DATA_BLOCK "IMAC_MOTOR3_RECORD"
TITLE =  MOTOR3_RECORD
AUTHOR : HottendU
FAMILY : IMAC
VERSION : 0.2


  STRUCT
   MOTOR3_No001 : STRUCT
    System : WORD ;
    CmdOS : WORD ;
    MirrorCmdOS : WORD ;
    Test : WORD ;
    AlarmOS : WORD ;
    StatusOS : WORD ;
    SysStatusOS : WORD ;
    Status1 : WORD ;
    Status2 : WORD ;
    Status3 : BYTE ;
    InputEdges : BYTE ;
    AutoEdges : WORD ;
    DataTimeExtFault : STRUCT
     StartTime : DINT ;
     StartEdge : BOOL ;
    END_STRUCT ;
    DataTimeFeedback : STRUCT
     StartTime : DINT ;
     StartEdge : BOOL ;
    END_STRUCT ;
    DataTimeActFault : STRUCT
     StartTime : DINT ;
     StartEdge : BOOL ;
    END_STRUCT ;
    DataTimeAutoAl : STRUCT
     StartTime : DINT ;
     StartEdge : BOOL ;
    END_STRUCT ;
    DataTimeRestart : STRUCT
     StartTime : DINT ;
     StartEdge : BOOL ;
    END_STRUCT ;
    DataTimeChgSF : STRUCT
     StartTime : DINT ;
     StartEdge : BOOL ;
    END_STRUCT ;
    DataTimeChgFS : STRUCT
     StartTime : DINT ;
     StartEdge : BOOL ;
    END_STRUCT ;
    DataTimeChgDirec : STRUCT
     StartTime : DINT ;
     StartEdge : BOOL ;
    END_STRUCT ;
    PCONF : STRUCT 	//// PCONF MOTOR3 - Instance 001
     Modeswitches : STRUCT
      M0_ConstantOut : BOOL  := TRUE;	// Constant Output MST1 MST2 MSTO (1); Feedback depended Output Anst. (0)
      M1_AutoManLoc : BOOL  := TRUE;	// AUTO/ MANUAL/ LOCAL (1); MANUAL/ LOCAL (0)
      M2_NoActFeedFault : BOOL ;	// No Action- and Non-Feedback fault(1),
      M3_NoStopIfFault : BOOL  := TRUE;	// No Stop-Signal if Failure occurs (1)
      M4_RestrtAftBlack : BOOL  := TRUE;	// Restart after Blackout (1)
      M5_ResetOSonly : BOOL  := TRUE;	// Reset Alarm only with RESET from OS (1); RESET and START/STOP-Command (0)
      sw06 : BOOL ;
      M7_ChgSFviaStop : BOOL ;	// Change from Slow->Fast via STOP(1)
      M8_ChgFSviaStop : BOOL ;	// Change from Fast->Slow via STOP(1)
      M9_StopIfAutoFail : BOOL ;	// Direct Stop if Auto Failure (1)
      M10_ExtFaultNC : BOOL ;	// External Fault is NC (1)
      sw11 : BOOL ;
      sw12 : BOOL ;
      sw13 : BOOL ;
      sw14 : BOOL ;
      sw15 : BOOL ;	//
     END_STRUCT ;
     DlyTExtFault : TIME  := T#1S;	// Setpoint external fault delay
     DlyTFeedback : TIME  := T#1S;	// Setpoint feedback fault delay
     DlyTActFault : TIME  := T#5S;	// Setpoint Action Fault delay
     DlyTAutoAl : TIME  := T#1S;	// Setpoint auto alarm delay
     DlyTRestart : TIME  := T#40S;	// Setpoint restart after blackout delay
     DlyTChgSF : TIME  := T#1S;	// Setpoint Waiting Delay Slow->Fast
     DlyTChgFS : TIME  := T#2S;	// Setpoint Waiting Delay Fast->Slow
     DlyTChgDirec : TIME  := T#4S;	// Setpoint change direction
    END_STRUCT ;
   END_STRUCT ;
   MOTOR3_No002 : STRUCT
    System : WORD ;
    CmdOS : WORD ;
    MirrorCmdOS : WORD ;
    Test : WORD ;
    AlarmOS : WORD ;
    StatusOS : WORD ;
    SysStatusOS : WORD ;
    Status1 : WORD ;
    Status2 : WORD ;
    Status3 : BYTE ;
    InputEdges : BYTE ;
    AutoEdges : WORD ;
    DataTimeExtFault : STRUCT
     StartTime : DINT ;
     StartEdge : BOOL ;
    END_STRUCT ;
    DataTimeFeedback : STRUCT
     StartTime : DINT ;
     StartEdge : BOOL ;
    END_STRUCT ;
    DataTimeActFault : STRUCT
     StartTime : DINT ;
     StartEdge : BOOL ;
    END_STRUCT ;
    DataTimeAutoAl : STRUCT
     StartTime : DINT ;
     StartEdge : BOOL ;
    END_STRUCT ;
    DataTimeRestart : STRUCT
     StartTime : DINT ;
     StartEdge : BOOL ;
    END_STRUCT ;
    DataTimeChgSF : STRUCT
     StartTime : DINT ;
     StartEdge : BOOL ;
    END_STRUCT ;
    DataTimeChgFS : STRUCT
     StartTime : DINT ;
     StartEdge : BOOL ;
    END_STRUCT ;
    DataTimeChgDirec : STRUCT
     StartTime : DINT ;
     StartEdge : BOOL ;
    END_STRUCT ;
    PCONF : STRUCT 	//// PCONF MOTOR3 - Instance 002
     Modeswitches : STRUCT
      M0_ConstantOut : BOOL ;	// Constant Output MST1 MST2 MSTO (1); Feedback depended Output Anst. (0)
      M1_AutoManLoc : BOOL ;	// AUTO/ MANUAL/ LOCAL (1); MANUAL/ LOCAL (0)
      M2_NoActFeedFault : BOOL ;	// No Action- and Non-Feedback fault(1),
      M3_NoStopIfFault : BOOL ;	// No Stop-Signal if Failure occurs (1)
      M4_RestrtAftBlack : BOOL ;	// Restart after Blackout (1)
      M5_ResetOSonly : BOOL ;	// Reset Alarm only with RESET from OS (1); RESET and START/STOP-Command (0)
      sw06 : BOOL ;
      M7_ChgSFviaStop : BOOL ;	// Change from Slow->Fast via STOP(1)
      M8_ChgFSviaStop : BOOL ;	// Change from Fast->Slow via STOP(1)
      M9_StopIfAutoFail : BOOL ;	// Direct Stop if Auto Failure (1)
      M10_ExtFaultNC : BOOL ;	// External Fault is NC (1)
      sw11 : BOOL ;
      sw12 : BOOL ;
      sw13 : BOOL ;
      sw14 : BOOL ;
      sw15 : BOOL ;	//
     END_STRUCT ;
     DlyTExtFault : TIME ;	// Setpoint external fault delay
     DlyTFeedback : TIME ;	// Setpoint feedback fault delay
     DlyTActFault : TIME ;	// Setpoint Action Fault delay
     DlyTAutoAl : TIME ;	// Setpoint auto alarm delay
     DlyTRestart : TIME ;	// Setpoint restart after blackout delay
     DlyTChgSF : TIME ;	// Setpoint Waiting Delay Slow->Fast
     DlyTChgFS : TIME ;	// Setpoint Waiting Delay Fast->Slow
     DlyTChgDirec : TIME ;	// Setpoint change direction
    END_STRUCT ;
   END_STRUCT ;
   MOTOR3_No003 : STRUCT
    System : WORD ;
    CmdOS : WORD ;
    MirrorCmdOS : WORD ;
    Test : WORD ;
    AlarmOS : WORD ;
    StatusOS : WORD ;
    SysStatusOS : WORD ;
    Status1 : WORD ;
    Status2 : WORD ;
    Status3 : BYTE ;
    InputEdges : BYTE ;
    AutoEdges : WORD ;
    DataTimeExtFault : STRUCT
     StartTime : DINT ;
     StartEdge : BOOL ;
    END_STRUCT ;
    DataTimeFeedback : STRUCT
     StartTime : DINT ;
     StartEdge : BOOL ;
    END_STRUCT ;
    DataTimeActFault : STRUCT
     StartTime : DINT ;
     StartEdge : BOOL ;
    END_STRUCT ;
    DataTimeAutoAl : STRUCT
     StartTime : DINT ;
     StartEdge : BOOL ;
    END_STRUCT ;
    DataTimeRestart : STRUCT
     StartTime : DINT ;
     StartEdge : BOOL ;
    END_STRUCT ;
    DataTimeChgSF : STRUCT
     StartTime : DINT ;
     StartEdge : BOOL ;
    END_STRUCT ;
    DataTimeChgFS : STRUCT
     StartTime : DINT ;
     StartEdge : BOOL ;
    END_STRUCT ;
    DataTimeChgDirec : STRUCT
     StartTime : DINT ;
     StartEdge : BOOL ;
    END_STRUCT ;
    PCONF : STRUCT 	//// PCONF MOTOR3 - Instance 003
     Modeswitches : STRUCT
      M0_ConstantOut : BOOL ;	// Constant Output MST1 MST2 MSTO (1); Feedback depended Output Anst. (0)
      M1_AutoManLoc : BOOL ;	// AUTO/ MANUAL/ LOCAL (1); MANUAL/ LOCAL (0)
      M2_NoActFeedFault : BOOL ;	// No Action- and Non-Feedback fault(1),
      M3_NoStopIfFault : BOOL ;	// No Stop-Signal if Failure occurs (1)
      M4_RestrtAftBlack : BOOL ;	// Restart after Blackout (1)
      M5_ResetOSonly : BOOL ;	// Reset Alarm only with RESET from OS (1); RESET and START/STOP-Command (0)
      sw06 : BOOL ;
      M7_ChgSFviaStop : BOOL ;	// Change from Slow->Fast via STOP(1)
      M8_ChgFSviaStop : BOOL ;	// Change from Fast->Slow via STOP(1)
      M9_StopIfAutoFail : BOOL ;	// Direct Stop if Auto Failure (1)
      M10_ExtFaultNC : BOOL ;	// External Fault is NC (1)
      sw11 : BOOL ;
      sw12 : BOOL ;
      sw13 : BOOL ;
      sw14 : BOOL ;
      sw15 : BOOL ;	//
     END_STRUCT ;
     DlyTExtFault : TIME ;	// Setpoint external fault delay
     DlyTFeedback : TIME ;	// Setpoint feedback fault delay
     DlyTActFault : TIME ;	// Setpoint Action Fault delay
     DlyTAutoAl : TIME ;	// Setpoint auto alarm delay
     DlyTRestart : TIME ;	// Setpoint restart after blackout delay
     DlyTChgSF : TIME ;	// Setpoint Waiting Delay Slow->Fast
     DlyTChgFS : TIME ;	// Setpoint Waiting Delay Fast->Slow
     DlyTChgDirec : TIME ;	// Setpoint change direction
    END_STRUCT ;
   END_STRUCT ;
   MOTOR3_No004 : STRUCT
    System : WORD ;
    CmdOS : WORD ;
    MirrorCmdOS : WORD ;
    Test : WORD ;
    AlarmOS : WORD ;
    StatusOS : WORD ;
    SysStatusOS : WORD ;
    Status1 : WORD ;
    Status2 : WORD ;
    Status3 : BYTE ;
    InputEdges : BYTE ;
    AutoEdges : WORD ;
    DataTimeExtFault : STRUCT
     StartTime : DINT ;
     StartEdge : BOOL ;
    END_STRUCT ;
    DataTimeFeedback : STRUCT
     StartTime : DINT ;
     StartEdge : BOOL ;
    END_STRUCT ;
    DataTimeActFault : STRUCT
     StartTime : DINT ;
     StartEdge : BOOL ;
    END_STRUCT ;
    DataTimeAutoAl : STRUCT
     StartTime : DINT ;
     StartEdge : BOOL ;
    END_STRUCT ;
    DataTimeRestart : STRUCT
     StartTime : DINT ;
     StartEdge : BOOL ;
    END_STRUCT ;
    DataTimeChgSF : STRUCT
     StartTime : DINT ;
     StartEdge : BOOL ;
    END_STRUCT ;
    DataTimeChgFS : STRUCT
     StartTime : DINT ;
     StartEdge : BOOL ;
    END_STRUCT ;
    DataTimeChgDirec : STRUCT
     StartTime : DINT ;
     StartEdge : BOOL ;
    END_STRUCT ;
    PCONF : STRUCT 	//// PCONF MOTOR3 - Instance 004
     Modeswitches : STRUCT
      M0_ConstantOut : BOOL ;	// Constant Output MST1 MST2 MSTO (1); Feedback depended Output Anst. (0)
      M1_AutoManLoc : BOOL ;	// AUTO/ MANUAL/ LOCAL (1); MANUAL/ LOCAL (0)
      M2_NoActFeedFault : BOOL ;	// No Action- and Non-Feedback fault(1),
      M3_NoStopIfFault : BOOL ;	// No Stop-Signal if Failure occurs (1)
      M4_RestrtAftBlack : BOOL ;	// Restart after Blackout (1)
      M5_ResetOSonly : BOOL ;	// Reset Alarm only with RESET from OS (1); RESET and START/STOP-Command (0)
      sw06 : BOOL ;
      M7_ChgSFviaStop : BOOL ;	// Change from Slow->Fast via STOP(1)
      M8_ChgFSviaStop : BOOL ;	// Change from Fast->Slow via STOP(1)
      M9_StopIfAutoFail : BOOL ;	// Direct Stop if Auto Failure (1)
      M10_ExtFaultNC : BOOL ;	// External Fault is NC (1)
      sw11 : BOOL ;
      sw12 : BOOL ;
      sw13 : BOOL ;
      sw14 : BOOL ;
      sw15 : BOOL ;	//
     END_STRUCT ;
     DlyTExtFault : TIME ;	// Setpoint external fault delay
     DlyTFeedback : TIME ;	// Setpoint feedback fault delay
     DlyTActFault : TIME ;	// Setpoint Action Fault delay
     DlyTAutoAl : TIME ;	// Setpoint auto alarm delay
     DlyTRestart : TIME ;	// Setpoint restart after blackout delay
     DlyTChgSF : TIME ;	// Setpoint Waiting Delay Slow->Fast
     DlyTChgFS : TIME ;	// Setpoint Waiting Delay Fast->Slow
     DlyTChgDirec : TIME ;	// Setpoint change direction
    END_STRUCT ;
   END_STRUCT ;
   MOTOR3_No005 : STRUCT
    System : WORD ;
    CmdOS : WORD ;
    MirrorCmdOS : WORD ;
    Test : WORD ;
    AlarmOS : WORD ;
    StatusOS : WORD ;
    SysStatusOS : WORD ;
    Status1 : WORD ;
    Status2 : WORD ;
    Status3 : BYTE ;
    InputEdges : BYTE ;
    AutoEdges : WORD ;
    DataTimeExtFault : STRUCT
     StartTime : DINT ;
     StartEdge : BOOL ;
    END_STRUCT ;
    DataTimeFeedback : STRUCT
     StartTime : DINT ;
     StartEdge : BOOL ;
    END_STRUCT ;
    DataTimeActFault : STRUCT
     StartTime : DINT ;
     StartEdge : BOOL ;
    END_STRUCT ;
    DataTimeAutoAl : STRUCT
     StartTime : DINT ;
     StartEdge : BOOL ;
    END_STRUCT ;
    DataTimeRestart : STRUCT
     StartTime : DINT ;
     StartEdge : BOOL ;
    END_STRUCT ;
    DataTimeChgSF : STRUCT
     StartTime : DINT ;
     StartEdge : BOOL ;
    END_STRUCT ;
    DataTimeChgFS : STRUCT
     StartTime : DINT ;
     StartEdge : BOOL ;
    END_STRUCT ;
    DataTimeChgDirec : STRUCT
     StartTime : DINT ;
     StartEdge : BOOL ;
    END_STRUCT ;
    PCONF : STRUCT 	//// PCONF MOTOR3 - Instance 005
     Modeswitches : STRUCT
      M0_ConstantOut : BOOL ;	// Constant Output MST1 MST2 MSTO (1); Feedback depended Output Anst. (0)
      M1_AutoManLoc : BOOL ;	// AUTO/ MANUAL/ LOCAL (1); MANUAL/ LOCAL (0)
      M2_NoActFeedFault : BOOL ;	// No Action- and Non-Feedback fault(1),
      M3_NoStopIfFault : BOOL ;	// No Stop-Signal if Failure occurs (1)
      M4_RestrtAftBlack : BOOL ;	// Restart after Blackout (1)
      M5_ResetOSonly : BOOL ;	// Reset Alarm only with RESET from OS (1); RESET and START/STOP-Command (0)
      sw06 : BOOL ;
      M7_ChgSFviaStop : BOOL ;	// Change from Slow->Fast via STOP(1)
      M8_ChgFSviaStop : BOOL ;	// Change from Fast->Slow via STOP(1)
      M9_StopIfAutoFail : BOOL ;	// Direct Stop if Auto Failure (1)
      M10_ExtFaultNC : BOOL ;	// External Fault is NC (1)
      sw11 : BOOL ;
      sw12 : BOOL ;
      sw13 : BOOL ;
      sw14 : BOOL ;
      sw15 : BOOL ;	//
     END_STRUCT ;
     DlyTExtFault : TIME ;	// Setpoint external fault delay
     DlyTFeedback : TIME ;	// Setpoint feedback fault delay
     DlyTActFault : TIME ;	// Setpoint Action Fault delay
     DlyTAutoAl : TIME ;	// Setpoint auto alarm delay
     DlyTRestart : TIME ;	// Setpoint restart after blackout delay
     DlyTChgSF : TIME ;	// Setpoint Waiting Delay Slow->Fast
     DlyTChgFS : TIME ;	// Setpoint Waiting Delay Fast->Slow
     DlyTChgDirec : TIME ;	// Setpoint change direction
    END_STRUCT ;
   END_STRUCT ;
   MOTOR3_No006 : STRUCT
    System : WORD ;
    CmdOS : WORD ;
    MirrorCmdOS : WORD ;
    Test : WORD ;
    AlarmOS : WORD ;
    StatusOS : WORD ;
    SysStatusOS : WORD ;
    Status1 : WORD ;
    Status2 : WORD ;
    Status3 : BYTE ;
    InputEdges : BYTE ;
    AutoEdges : WORD ;
    DataTimeExtFault : STRUCT
     StartTime : DINT ;
     StartEdge : BOOL ;
    END_STRUCT ;
    DataTimeFeedback : STRUCT
     StartTime : DINT ;
     StartEdge : BOOL ;
    END_STRUCT ;
    DataTimeActFault : STRUCT
     StartTime : DINT ;
     StartEdge : BOOL ;
    END_STRUCT ;
    DataTimeAutoAl : STRUCT
     StartTime : DINT ;
     StartEdge : BOOL ;
    END_STRUCT ;
    DataTimeRestart : STRUCT
     StartTime : DINT ;
     StartEdge : BOOL ;
    END_STRUCT ;
    DataTimeChgSF : STRUCT
     StartTime : DINT ;
     StartEdge : BOOL ;
    END_STRUCT ;
    DataTimeChgFS : STRUCT
     StartTime : DINT ;
     StartEdge : BOOL ;
    END_STRUCT ;
    DataTimeChgDirec : STRUCT
     StartTime : DINT ;
     StartEdge : BOOL ;
    END_STRUCT ;
    PCONF : STRUCT 	//// PCONF MOTOR3 - Instance 006
     Modeswitches : STRUCT
      M0_ConstantOut : BOOL ;	// Constant Output MST1 MST2 MSTO (1); Feedback depended Output Anst. (0)
      M1_AutoManLoc : BOOL ;	// AUTO/ MANUAL/ LOCAL (1); MANUAL/ LOCAL (0)
      M2_NoActFeedFault : BOOL ;	// No Action- and Non-Feedback fault(1),
      M3_NoStopIfFault : BOOL ;	// No Stop-Signal if Failure occurs (1)
      M4_RestrtAftBlack : BOOL ;	// Restart after Blackout (1)
      M5_ResetOSonly : BOOL ;	// Reset Alarm only with RESET from OS (1); RESET and START/STOP-Command (0)
      sw06 : BOOL ;
      M7_ChgSFviaStop : BOOL ;	// Change from Slow->Fast via STOP(1)
      M8_ChgFSviaStop : BOOL ;	// Change from Fast->Slow via STOP(1)
      M9_StopIfAutoFail : BOOL ;	// Direct Stop if Auto Failure (1)
      M10_ExtFaultNC : BOOL ;	// External Fault is NC (1)
      sw11 : BOOL ;
      sw12 : BOOL ;
      sw13 : BOOL ;
      sw14 : BOOL ;
      sw15 : BOOL ;	//
     END_STRUCT ;
     DlyTExtFault : TIME ;	// Setpoint external fault delay
     DlyTFeedback : TIME ;	// Setpoint feedback fault delay
     DlyTActFault : TIME ;	// Setpoint Action Fault delay
     DlyTAutoAl : TIME ;	// Setpoint auto alarm delay
     DlyTRestart : TIME ;	// Setpoint restart after blackout delay
     DlyTChgSF : TIME ;	// Setpoint Waiting Delay Slow->Fast
     DlyTChgFS : TIME ;	// Setpoint Waiting Delay Fast->Slow
     DlyTChgDirec : TIME ;	// Setpoint change direction
    END_STRUCT ;
   END_STRUCT ;
   MOTOR3_No007 : STRUCT
    System : WORD ;
    CmdOS : WORD ;
    MirrorCmdOS : WORD ;
    Test : WORD ;
    AlarmOS : WORD ;
    StatusOS : WORD ;
    SysStatusOS : WORD ;
    Status1 : WORD ;
    Status2 : WORD ;
    Status3 : BYTE ;
    InputEdges : BYTE ;
    AutoEdges : WORD ;
    DataTimeExtFault : STRUCT
     StartTime : DINT ;
     StartEdge : BOOL ;
    END_STRUCT ;
    DataTimeFeedback : STRUCT
     StartTime : DINT ;
     StartEdge : BOOL ;
    END_STRUCT ;
    DataTimeActFault : STRUCT
     StartTime : DINT ;
     StartEdge : BOOL ;
    END_STRUCT ;
    DataTimeAutoAl : STRUCT
     StartTime : DINT ;
     StartEdge : BOOL ;
    END_STRUCT ;
    DataTimeRestart : STRUCT
     StartTime : DINT ;
     StartEdge : BOOL ;
    END_STRUCT ;
    DataTimeChgSF : STRUCT
     StartTime : DINT ;
     StartEdge : BOOL ;
    END_STRUCT ;
    DataTimeChgFS : STRUCT
     StartTime : DINT ;
     StartEdge : BOOL ;
    END_STRUCT ;
    DataTimeChgDirec : STRUCT
     StartTime : DINT ;
     StartEdge : BOOL ;
    END_STRUCT ;
    PCONF : STRUCT 	//// PCONF MOTOR3 - Instance 007
     Modeswitches : STRUCT
      M0_ConstantOut : BOOL ;	// Constant Output MST1 MST2 MSTO (1); Feedback depended Output Anst. (0)
      M1_AutoManLoc : BOOL ;	// AUTO/ MANUAL/ LOCAL (1); MANUAL/ LOCAL (0)
      M2_NoActFeedFault : BOOL ;	// No Action- and Non-Feedback fault(1),
      M3_NoStopIfFault : BOOL ;	// No Stop-Signal if Failure occurs (1)
      M4_RestrtAftBlack : BOOL ;	// Restart after Blackout (1)
      M5_ResetOSonly : BOOL ;	// Reset Alarm only with RESET from OS (1); RESET and START/STOP-Command (0)
      sw06 : BOOL ;
      M7_ChgSFviaStop : BOOL ;	// Change from Slow->Fast via STOP(1)
      M8_ChgFSviaStop : BOOL ;	// Change from Fast->Slow via STOP(1)
      M9_StopIfAutoFail : BOOL ;	// Direct Stop if Auto Failure (1)
      M10_ExtFaultNC : BOOL ;	// External Fault is NC (1)
      sw11 : BOOL ;
      sw12 : BOOL ;
      sw13 : BOOL ;
      sw14 : BOOL ;
      sw15 : BOOL ;	//
     END_STRUCT ;
     DlyTExtFault : TIME ;	// Setpoint external fault delay
     DlyTFeedback : TIME ;	// Setpoint feedback fault delay
     DlyTActFault : TIME ;	// Setpoint Action Fault delay
     DlyTAutoAl : TIME ;	// Setpoint auto alarm delay
     DlyTRestart : TIME ;	// Setpoint restart after blackout delay
     DlyTChgSF : TIME ;	// Setpoint Waiting Delay Slow->Fast
     DlyTChgFS : TIME ;	// Setpoint Waiting Delay Fast->Slow
     DlyTChgDirec : TIME ;	// Setpoint change direction
    END_STRUCT ;
   END_STRUCT ;
   MOTOR3_No008 : STRUCT
    System : WORD ;
    CmdOS : WORD ;
    MirrorCmdOS : WORD ;
    Test : WORD ;
    AlarmOS : WORD ;
    StatusOS : WORD ;
    SysStatusOS : WORD ;
    Status1 : WORD ;
    Status2 : WORD ;
    Status3 : BYTE ;
    InputEdges : BYTE ;
    AutoEdges : WORD ;
    DataTimeExtFault : STRUCT
     StartTime : DINT ;
     StartEdge : BOOL ;
    END_STRUCT ;
    DataTimeFeedback : STRUCT
     StartTime : DINT ;
     StartEdge : BOOL ;
    END_STRUCT ;
    DataTimeActFault : STRUCT
     StartTime : DINT ;
     StartEdge : BOOL ;
    END_STRUCT ;
    DataTimeAutoAl : STRUCT
     StartTime : DINT ;
     StartEdge : BOOL ;
    END_STRUCT ;
    DataTimeRestart : STRUCT
     StartTime : DINT ;
     StartEdge : BOOL ;
    END_STRUCT ;
    DataTimeChgSF : STRUCT
     StartTime : DINT ;
     StartEdge : BOOL ;
    END_STRUCT ;
    DataTimeChgFS : STRUCT
     StartTime : DINT ;
     StartEdge : BOOL ;
    END_STRUCT ;
    DataTimeChgDirec : STRUCT
     StartTime : DINT ;
     StartEdge : BOOL ;
    END_STRUCT ;
    PCONF : STRUCT 	//// PCONF MOTOR3 - Instance 008
     Modeswitches : STRUCT
      M0_ConstantOut : BOOL ;	// Constant Output MST1 MST2 MSTO (1); Feedback depended Output Anst. (0)
      M1_AutoManLoc : BOOL ;	// AUTO/ MANUAL/ LOCAL (1); MANUAL/ LOCAL (0)
      M2_NoActFeedFault : BOOL ;	// No Action- and Non-Feedback fault(1),
      M3_NoStopIfFault : BOOL ;	// No Stop-Signal if Failure occurs (1)
      M4_RestrtAftBlack : BOOL ;	// Restart after Blackout (1)
      M5_ResetOSonly : BOOL ;	// Reset Alarm only with RESET from OS (1); RESET and START/STOP-Command (0)
      sw06 : BOOL ;
      M7_ChgSFviaStop : BOOL ;	// Change from Slow->Fast via STOP(1)
      M8_ChgFSviaStop : BOOL ;	// Change from Fast->Slow via STOP(1)
      M9_StopIfAutoFail : BOOL ;	// Direct Stop if Auto Failure (1)
      M10_ExtFaultNC : BOOL ;	// External Fault is NC (1)
      sw11 : BOOL ;
      sw12 : BOOL ;
      sw13 : BOOL ;
      sw14 : BOOL ;
      sw15 : BOOL ;	//
     END_STRUCT ;
     DlyTExtFault : TIME ;	// Setpoint external fault delay
     DlyTFeedback : TIME ;	// Setpoint feedback fault delay
     DlyTActFault : TIME ;	// Setpoint Action Fault delay
     DlyTAutoAl : TIME ;	// Setpoint auto alarm delay
     DlyTRestart : TIME ;	// Setpoint restart after blackout delay
     DlyTChgSF : TIME ;	// Setpoint Waiting Delay Slow->Fast
     DlyTChgFS : TIME ;	// Setpoint Waiting Delay Fast->Slow
     DlyTChgDirec : TIME ;	// Setpoint change direction
    END_STRUCT ;
   END_STRUCT ;
   MOTOR3_No009 : STRUCT
    System : WORD ;
    CmdOS : WORD ;
    MirrorCmdOS : WORD ;
    Test : WORD ;
    AlarmOS : WORD ;
    StatusOS : WORD ;
    SysStatusOS : WORD ;
    Status1 : WORD ;
    Status2 : WORD ;
    Status3 : BYTE ;
    InputEdges : BYTE ;
    AutoEdges : WORD ;
    DataTimeExtFault : STRUCT
     StartTime : DINT ;
     StartEdge : BOOL ;
    END_STRUCT ;
    DataTimeFeedback : STRUCT
     StartTime : DINT ;
     StartEdge : BOOL ;
    END_STRUCT ;
    DataTimeActFault : STRUCT
     StartTime : DINT ;
     StartEdge : BOOL ;
    END_STRUCT ;
    DataTimeAutoAl : STRUCT
     StartTime : DINT ;
     StartEdge : BOOL ;
    END_STRUCT ;
    DataTimeRestart : STRUCT
     StartTime : DINT ;
     StartEdge : BOOL ;
    END_STRUCT ;
    DataTimeChgSF : STRUCT
     StartTime : DINT ;
     StartEdge : BOOL ;
    END_STRUCT ;
    DataTimeChgFS : STRUCT
     StartTime : DINT ;
     StartEdge : BOOL ;
    END_STRUCT ;
    DataTimeChgDirec : STRUCT
     StartTime : DINT ;
     StartEdge : BOOL ;
    END_STRUCT ;
    PCONF : STRUCT 	//// PCONF MOTOR3 - Instance 009
     Modeswitches : STRUCT
      M0_ConstantOut : BOOL ;	// Constant Output MST1 MST2 MSTO (1); Feedback depended Output Anst. (0)
      M1_AutoManLoc : BOOL ;	// AUTO/ MANUAL/ LOCAL (1); MANUAL/ LOCAL (0)
      M2_NoActFeedFault : BOOL ;	// No Action- and Non-Feedback fault(1),
      M3_NoStopIfFault : BOOL ;	// No Stop-Signal if Failure occurs (1)
      M4_RestrtAftBlack : BOOL ;	// Restart after Blackout (1)
      M5_ResetOSonly : BOOL ;	// Reset Alarm only with RESET from OS (1); RESET and START/STOP-Command (0)
      sw06 : BOOL ;
      M7_ChgSFviaStop : BOOL ;	// Change from Slow->Fast via STOP(1)
      M8_ChgFSviaStop : BOOL ;	// Change from Fast->Slow via STOP(1)
      M9_StopIfAutoFail : BOOL ;	// Direct Stop if Auto Failure (1)
      M10_ExtFaultNC : BOOL ;	// External Fault is NC (1)
      sw11 : BOOL ;
      sw12 : BOOL ;
      sw13 : BOOL ;
      sw14 : BOOL ;
      sw15 : BOOL ;	//
     END_STRUCT ;
     DlyTExtFault : TIME ;	// Setpoint external fault delay
     DlyTFeedback : TIME ;	// Setpoint feedback fault delay
     DlyTActFault : TIME ;	// Setpoint Action Fault delay
     DlyTAutoAl : TIME ;	// Setpoint auto alarm delay
     DlyTRestart : TIME ;	// Setpoint restart after blackout delay
     DlyTChgSF : TIME ;	// Setpoint Waiting Delay Slow->Fast
     DlyTChgFS : TIME ;	// Setpoint Waiting Delay Fast->Slow
     DlyTChgDirec : TIME ;	// Setpoint change direction
    END_STRUCT ;
   END_STRUCT ;
   MOTOR3_No010 : STRUCT
    System : WORD ;
    CmdOS : WORD ;
    MirrorCmdOS : WORD ;
    Test : WORD ;
    AlarmOS : WORD ;
    StatusOS : WORD ;
    SysStatusOS : WORD ;
    Status1 : WORD ;
    Status2 : WORD ;
    Status3 : BYTE ;
    InputEdges : BYTE ;
    AutoEdges : WORD ;
    DataTimeExtFault : STRUCT
     StartTime : DINT ;
     StartEdge : BOOL ;
    END_STRUCT ;
    DataTimeFeedback : STRUCT
     StartTime : DINT ;
     StartEdge : BOOL ;
    END_STRUCT ;
    DataTimeActFault : STRUCT
     StartTime : DINT ;
     StartEdge : BOOL ;
    END_STRUCT ;
    DataTimeAutoAl : STRUCT
     StartTime : DINT ;
     StartEdge : BOOL ;
    END_STRUCT ;
    DataTimeRestart : STRUCT
     StartTime : DINT ;
     StartEdge : BOOL ;
    END_STRUCT ;
    DataTimeChgSF : STRUCT
     StartTime : DINT ;
     StartEdge : BOOL ;
    END_STRUCT ;
    DataTimeChgFS : STRUCT
     StartTime : DINT ;
     StartEdge : BOOL ;
    END_STRUCT ;
    DataTimeChgDirec : STRUCT
     StartTime : DINT ;
     StartEdge : BOOL ;
    END_STRUCT ;
    PCONF : STRUCT 	//// PCONF MOTOR3 - Instance 010
     Modeswitches : STRUCT
      M0_ConstantOut : BOOL ;	// Constant Output MST1 MST2 MSTO (1); Feedback depended Output Anst. (0)
      M1_AutoManLoc : BOOL ;	// AUTO/ MANUAL/ LOCAL (1); MANUAL/ LOCAL (0)
      M2_NoActFeedFault : BOOL ;	// No Action- and Non-Feedback fault(1),
      M3_NoStopIfFault : BOOL ;	// No Stop-Signal if Failure occurs (1)
      M4_RestrtAftBlack : BOOL ;	// Restart after Blackout (1)
      M5_ResetOSonly : BOOL ;	// Reset Alarm only with RESET from OS (1); RESET and START/STOP-Command (0)
      sw06 : BOOL ;
      M7_ChgSFviaStop : BOOL ;	// Change from Slow->Fast via STOP(1)
      M8_ChgFSviaStop : BOOL ;	// Change from Fast->Slow via STOP(1)
      M9_StopIfAutoFail : BOOL ;	// Direct Stop if Auto Failure (1)
      M10_ExtFaultNC : BOOL ;	// External Fault is NC (1)
      sw11 : BOOL ;
      sw12 : BOOL ;
      sw13 : BOOL ;
      sw14 : BOOL ;
      sw15 : BOOL ;	//
     END_STRUCT ;
     DlyTExtFault : TIME ;	// Setpoint external fault delay
     DlyTFeedback : TIME ;	// Setpoint feedback fault delay
     DlyTActFault : TIME ;	// Setpoint Action Fault delay
     DlyTAutoAl : TIME ;	// Setpoint auto alarm delay
     DlyTRestart : TIME ;	// Setpoint restart after blackout delay
     DlyTChgSF : TIME ;	// Setpoint Waiting Delay Slow->Fast
     DlyTChgFS : TIME ;	// Setpoint Waiting Delay Fast->Slow
     DlyTChgDirec : TIME ;	// Setpoint change direction
    END_STRUCT ;
   END_STRUCT ;
   MOTOR3_No011 : STRUCT
    System : WORD ;
    CmdOS : WORD ;
    MirrorCmdOS : WORD ;
    Test : WORD ;
    AlarmOS : WORD ;
    StatusOS : WORD ;
    SysStatusOS : WORD ;
    Status1 : WORD ;
    Status2 : WORD ;
    Status3 : BYTE ;
    InputEdges : BYTE ;
    AutoEdges : WORD ;
    DataTimeExtFault : STRUCT
     StartTime : DINT ;
     StartEdge : BOOL ;
    END_STRUCT ;
    DataTimeFeedback : STRUCT
     StartTime : DINT ;
     StartEdge : BOOL ;
    END_STRUCT ;
    DataTimeActFault : STRUCT
     StartTime : DINT ;
     StartEdge : BOOL ;
    END_STRUCT ;
    DataTimeAutoAl : STRUCT
     StartTime : DINT ;
     StartEdge : BOOL ;
    END_STRUCT ;
    DataTimeRestart : STRUCT
     StartTime : DINT ;
     StartEdge : BOOL ;
    END_STRUCT ;
    DataTimeChgSF : STRUCT
     StartTime : DINT ;
     StartEdge : BOOL ;
    END_STRUCT ;
    DataTimeChgFS : STRUCT
     StartTime : DINT ;
     StartEdge : BOOL ;
    END_STRUCT ;
    DataTimeChgDirec : STRUCT
     StartTime : DINT ;
     StartEdge : BOOL ;
    END_STRUCT ;
    PCONF : STRUCT 	//// PCONF MOTOR3 - Instance 011
     Modeswitches : STRUCT
      M0_ConstantOut : BOOL ;	// Constant Output MST1 MST2 MSTO (1); Feedback depended Output Anst. (0)
      M1_AutoManLoc : BOOL ;	// AUTO/ MANUAL/ LOCAL (1); MANUAL/ LOCAL (0)
      M2_NoActFeedFault : BOOL ;	// No Action- and Non-Feedback fault(1),
      M3_NoStopIfFault : BOOL ;	// No Stop-Signal if Failure occurs (1)
      M4_RestrtAftBlack : BOOL ;	// Restart after Blackout (1)
      M5_ResetOSonly : BOOL ;	// Reset Alarm only with RESET from OS (1); RESET and START/STOP-Command (0)
      sw06 : BOOL ;
      M7_ChgSFviaStop : BOOL ;	// Change from Slow->Fast via STOP(1)
      M8_ChgFSviaStop : BOOL ;	// Change from Fast->Slow via STOP(1)
      M9_StopIfAutoFail : BOOL ;	// Direct Stop if Auto Failure (1)
      M10_ExtFaultNC : BOOL ;	// External Fault is NC (1)
      sw11 : BOOL ;
      sw12 : BOOL ;
      sw13 : BOOL ;
      sw14 : BOOL ;
      sw15 : BOOL ;	//
     END_STRUCT ;
     DlyTExtFault : TIME ;	// Setpoint external fault delay
     DlyTFeedback : TIME ;	// Setpoint feedback fault delay
     DlyTActFault : TIME ;	// Setpoint Action Fault delay
     DlyTAutoAl : TIME ;	// Setpoint auto alarm delay
     DlyTRestart : TIME ;	// Setpoint restart after blackout delay
     DlyTChgSF : TIME ;	// Setpoint Waiting Delay Slow->Fast
     DlyTChgFS : TIME ;	// Setpoint Waiting Delay Fast->Slow
     DlyTChgDirec : TIME ;	// Setpoint change direction
    END_STRUCT ;
   END_STRUCT ;
   MOTOR3_No012 : STRUCT
    System : WORD ;
    CmdOS : WORD ;
    MirrorCmdOS : WORD ;
    Test : WORD ;
    AlarmOS : WORD ;
    StatusOS : WORD ;
    SysStatusOS : WORD ;
    Status1 : WORD ;
    Status2 : WORD ;
    Status3 : BYTE ;
    InputEdges : BYTE ;
    AutoEdges : WORD ;
    DataTimeExtFault : STRUCT
     StartTime : DINT ;
     StartEdge : BOOL ;
    END_STRUCT ;
    DataTimeFeedback : STRUCT
     StartTime : DINT ;
     StartEdge : BOOL ;
    END_STRUCT ;
    DataTimeActFault : STRUCT
     StartTime : DINT ;
     StartEdge : BOOL ;
    END_STRUCT ;
    DataTimeAutoAl : STRUCT
     StartTime : DINT ;
     StartEdge : BOOL ;
    END_STRUCT ;
    DataTimeRestart : STRUCT
     StartTime : DINT ;
     StartEdge : BOOL ;
    END_STRUCT ;
    DataTimeChgSF : STRUCT
     StartTime : DINT ;
     StartEdge : BOOL ;
    END_STRUCT ;
    DataTimeChgFS : STRUCT
     StartTime : DINT ;
     StartEdge : BOOL ;
    END_STRUCT ;
    DataTimeChgDirec : STRUCT
     StartTime : DINT ;
     StartEdge : BOOL ;
    END_STRUCT ;
    PCONF : STRUCT 	//// PCONF MOTOR3 - Instance 012
     Modeswitches : STRUCT
      M0_ConstantOut : BOOL ;	// Constant Output MST1 MST2 MSTO (1); Feedback depended Output Anst. (0)
      M1_AutoManLoc : BOOL ;	// AUTO/ MANUAL/ LOCAL (1); MANUAL/ LOCAL (0)
      M2_NoActFeedFault : BOOL ;	// No Action- and Non-Feedback fault(1),
      M3_NoStopIfFault : BOOL ;	// No Stop-Signal if Failure occurs (1)
      M4_RestrtAftBlack : BOOL ;	// Restart after Blackout (1)
      M5_ResetOSonly : BOOL ;	// Reset Alarm only with RESET from OS (1); RESET and START/STOP-Command (0)
      sw06 : BOOL ;
      M7_ChgSFviaStop : BOOL ;	// Change from Slow->Fast via STOP(1)
      M8_ChgFSviaStop : BOOL ;	// Change from Fast->Slow via STOP(1)
      M9_StopIfAutoFail : BOOL ;	// Direct Stop if Auto Failure (1)
      M10_ExtFaultNC : BOOL ;	// External Fault is NC (1)
      sw11 : BOOL ;
      sw12 : BOOL ;
      sw13 : BOOL ;
      sw14 : BOOL ;
      sw15 : BOOL ;	//
     END_STRUCT ;
     DlyTExtFault : TIME ;	// Setpoint external fault delay
     DlyTFeedback : TIME ;	// Setpoint feedback fault delay
     DlyTActFault : TIME ;	// Setpoint Action Fault delay
     DlyTAutoAl : TIME ;	// Setpoint auto alarm delay
     DlyTRestart : TIME ;	// Setpoint restart after blackout delay
     DlyTChgSF : TIME ;	// Setpoint Waiting Delay Slow->Fast
     DlyTChgFS : TIME ;	// Setpoint Waiting Delay Fast->Slow
     DlyTChgDirec : TIME ;	// Setpoint change direction
    END_STRUCT ;
   END_STRUCT ;
   MOTOR3_No013 : STRUCT
    System : WORD ;
    CmdOS : WORD ;
    MirrorCmdOS : WORD ;
    Test : WORD ;
    AlarmOS : WORD ;
    StatusOS : WORD ;
    SysStatusOS : WORD ;
    Status1 : WORD ;
    Status2 : WORD ;
    Status3 : BYTE ;
    InputEdges : BYTE ;
    AutoEdges : WORD ;
    DataTimeExtFault : STRUCT
     StartTime : DINT ;
     StartEdge : BOOL ;
    END_STRUCT ;
    DataTimeFeedback : STRUCT
     StartTime : DINT ;
     StartEdge : BOOL ;
    END_STRUCT ;
    DataTimeActFault : STRUCT
     StartTime : DINT ;
     StartEdge : BOOL ;
    END_STRUCT ;
    DataTimeAutoAl : STRUCT
     StartTime : DINT ;
     StartEdge : BOOL ;
    END_STRUCT ;
    DataTimeRestart : STRUCT
     StartTime : DINT ;
     StartEdge : BOOL ;
    END_STRUCT ;
    DataTimeChgSF : STRUCT
     StartTime : DINT ;
     StartEdge : BOOL ;
    END_STRUCT ;
    DataTimeChgFS : STRUCT
     StartTime : DINT ;
     StartEdge : BOOL ;
    END_STRUCT ;
    DataTimeChgDirec : STRUCT
     StartTime : DINT ;
     StartEdge : BOOL ;
    END_STRUCT ;
    PCONF : STRUCT 	//// PCONF MOTOR3 - Instance 013
     Modeswitches : STRUCT
      M0_ConstantOut : BOOL ;	// Constant Output MST1 MST2 MSTO (1); Feedback depended Output Anst. (0)
      M1_AutoManLoc : BOOL ;	// AUTO/ MANUAL/ LOCAL (1); MANUAL/ LOCAL (0)
      M2_NoActFeedFault : BOOL ;	// No Action- and Non-Feedback fault(1),
      M3_NoStopIfFault : BOOL ;	// No Stop-Signal if Failure occurs (1)
      M4_RestrtAftBlack : BOOL ;	// Restart after Blackout (1)
      M5_ResetOSonly : BOOL ;	// Reset Alarm only with RESET from OS (1); RESET and START/STOP-Command (0)
      sw06 : BOOL ;
      M7_ChgSFviaStop : BOOL ;	// Change from Slow->Fast via STOP(1)
      M8_ChgFSviaStop : BOOL ;	// Change from Fast->Slow via STOP(1)
      M9_StopIfAutoFail : BOOL ;	// Direct Stop if Auto Failure (1)
      M10_ExtFaultNC : BOOL ;	// External Fault is NC (1)
      sw11 : BOOL ;
      sw12 : BOOL ;
      sw13 : BOOL ;
      sw14 : BOOL ;
      sw15 : BOOL ;	//
     END_STRUCT ;
     DlyTExtFault : TIME ;	// Setpoint external fault delay
     DlyTFeedback : TIME ;	// Setpoint feedback fault delay
     DlyTActFault : TIME ;	// Setpoint Action Fault delay
     DlyTAutoAl : TIME ;	// Setpoint auto alarm delay
     DlyTRestart : TIME ;	// Setpoint restart after blackout delay
     DlyTChgSF : TIME ;	// Setpoint Waiting Delay Slow->Fast
     DlyTChgFS : TIME ;	// Setpoint Waiting Delay Fast->Slow
     DlyTChgDirec : TIME ;	// Setpoint change direction
    END_STRUCT ;
   END_STRUCT ;
   MOTOR3_No014 : STRUCT
    System : WORD ;
    CmdOS : WORD ;
    MirrorCmdOS : WORD ;
    Test : WORD ;
    AlarmOS : WORD ;
    StatusOS : WORD ;
    SysStatusOS : WORD ;
    Status1 : WORD ;
    Status2 : WORD ;
    Status3 : BYTE ;
    InputEdges : BYTE ;
    AutoEdges : WORD ;
    DataTimeExtFault : STRUCT
     StartTime : DINT ;
     StartEdge : BOOL ;
    END_STRUCT ;
    DataTimeFeedback : STRUCT
     StartTime : DINT ;
     StartEdge : BOOL ;
    END_STRUCT ;
    DataTimeActFault : STRUCT
     StartTime : DINT ;
     StartEdge : BOOL ;
    END_STRUCT ;
    DataTimeAutoAl : STRUCT
     StartTime : DINT ;
     StartEdge : BOOL ;
    END_STRUCT ;
    DataTimeRestart : STRUCT
     StartTime : DINT ;
     StartEdge : BOOL ;
    END_STRUCT ;
    DataTimeChgSF : STRUCT
     StartTime : DINT ;
     StartEdge : BOOL ;
    END_STRUCT ;
    DataTimeChgFS : STRUCT
     StartTime : DINT ;
     StartEdge : BOOL ;
    END_STRUCT ;
    DataTimeChgDirec : STRUCT
     StartTime : DINT ;
     StartEdge : BOOL ;
    END_STRUCT ;
    PCONF : STRUCT 	//// PCONF MOTOR3 - Instance 014
     Modeswitches : STRUCT
      M0_ConstantOut : BOOL ;	// Constant Output MST1 MST2 MSTO (1); Feedback depended Output Anst. (0)
      M1_AutoManLoc : BOOL ;	// AUTO/ MANUAL/ LOCAL (1); MANUAL/ LOCAL (0)
      M2_NoActFeedFault : BOOL ;	// No Action- and Non-Feedback fault(1),
      M3_NoStopIfFault : BOOL ;	// No Stop-Signal if Failure occurs (1)
      M4_RestrtAftBlack : BOOL ;	// Restart after Blackout (1)
      M5_ResetOSonly : BOOL ;	// Reset Alarm only with RESET from OS (1); RESET and START/STOP-Command (0)
      sw06 : BOOL ;
      M7_ChgSFviaStop : BOOL ;	// Change from Slow->Fast via STOP(1)
      M8_ChgFSviaStop : BOOL ;	// Change from Fast->Slow via STOP(1)
      M9_StopIfAutoFail : BOOL ;	// Direct Stop if Auto Failure (1)
      M10_ExtFaultNC : BOOL ;	// External Fault is NC (1)
      sw11 : BOOL ;
      sw12 : BOOL ;
      sw13 : BOOL ;
      sw14 : BOOL ;
      sw15 : BOOL ;	//
     END_STRUCT ;
     DlyTExtFault : TIME ;	// Setpoint external fault delay
     DlyTFeedback : TIME ;	// Setpoint feedback fault delay
     DlyTActFault : TIME ;	// Setpoint Action Fault delay
     DlyTAutoAl : TIME ;	// Setpoint auto alarm delay
     DlyTRestart : TIME ;	// Setpoint restart after blackout delay
     DlyTChgSF : TIME ;	// Setpoint Waiting Delay Slow->Fast
     DlyTChgFS : TIME ;	// Setpoint Waiting Delay Fast->Slow
     DlyTChgDirec : TIME ;	// Setpoint change direction
    END_STRUCT ;
   END_STRUCT ;
   MOTOR3_No015 : STRUCT
    System : WORD ;
    CmdOS : WORD ;
    MirrorCmdOS : WORD ;
    Test : WORD ;
    AlarmOS : WORD ;
    StatusOS : WORD ;
    SysStatusOS : WORD ;
    Status1 : WORD ;
    Status2 : WORD ;
    Status3 : BYTE ;
    InputEdges : BYTE ;
    AutoEdges : WORD ;
    DataTimeExtFault : STRUCT
     StartTime : DINT ;
     StartEdge : BOOL ;
    END_STRUCT ;
    DataTimeFeedback : STRUCT
     StartTime : DINT ;
     StartEdge : BOOL ;
    END_STRUCT ;
    DataTimeActFault : STRUCT
     StartTime : DINT ;
     StartEdge : BOOL ;
    END_STRUCT ;
    DataTimeAutoAl : STRUCT
     StartTime : DINT ;
     StartEdge : BOOL ;
    END_STRUCT ;
    DataTimeRestart : STRUCT
     StartTime : DINT ;
     StartEdge : BOOL ;
    END_STRUCT ;
    DataTimeChgSF : STRUCT
     StartTime : DINT ;
     StartEdge : BOOL ;
    END_STRUCT ;
    DataTimeChgFS : STRUCT
     StartTime : DINT ;
     StartEdge : BOOL ;
    END_STRUCT ;
    DataTimeChgDirec : STRUCT
     StartTime : DINT ;
     StartEdge : BOOL ;
    END_STRUCT ;
    PCONF : STRUCT 	//// PCONF MOTOR3 - Instance 015
     Modeswitches : STRUCT
      M0_ConstantOut : BOOL ;	// Constant Output MST1 MST2 MSTO (1); Feedback depended Output Anst. (0)
      M1_AutoManLoc : BOOL ;	// AUTO/ MANUAL/ LOCAL (1); MANUAL/ LOCAL (0)
      M2_NoActFeedFault : BOOL ;	// No Action- and Non-Feedback fault(1),
      M3_NoStopIfFault : BOOL ;	// No Stop-Signal if Failure occurs (1)
      M4_RestrtAftBlack : BOOL ;	// Restart after Blackout (1)
      M5_ResetOSonly : BOOL ;	// Reset Alarm only with RESET from OS (1); RESET and START/STOP-Command (0)
      sw06 : BOOL ;
      M7_ChgSFviaStop : BOOL ;	// Change from Slow->Fast via STOP(1)
      M8_ChgFSviaStop : BOOL ;	// Change from Fast->Slow via STOP(1)
      M9_StopIfAutoFail : BOOL ;	// Direct Stop if Auto Failure (1)
      M10_ExtFaultNC : BOOL ;	// External Fault is NC (1)
      sw11 : BOOL ;
      sw12 : BOOL ;
      sw13 : BOOL ;
      sw14 : BOOL ;
      sw15 : BOOL ;	//
     END_STRUCT ;
     DlyTExtFault : TIME ;	// Setpoint external fault delay
     DlyTFeedback : TIME ;	// Setpoint feedback fault delay
     DlyTActFault : TIME ;	// Setpoint Action Fault delay
     DlyTAutoAl : TIME ;	// Setpoint auto alarm delay
     DlyTRestart : TIME ;	// Setpoint restart after blackout delay
     DlyTChgSF : TIME ;	// Setpoint Waiting Delay Slow->Fast
     DlyTChgFS : TIME ;	// Setpoint Waiting Delay Fast->Slow
     DlyTChgDirec : TIME ;	// Setpoint change direction
    END_STRUCT ;
   END_STRUCT ;
   MOTOR3_No016 : STRUCT
    System : WORD ;
    CmdOS : WORD ;
    MirrorCmdOS : WORD ;
    Test : WORD ;
    AlarmOS : WORD ;
    StatusOS : WORD ;
    SysStatusOS : WORD ;
    Status1 : WORD ;
    Status2 : WORD ;
    Status3 : BYTE ;
    InputEdges : BYTE ;
    AutoEdges : WORD ;
    DataTimeExtFault : STRUCT
     StartTime : DINT ;
     StartEdge : BOOL ;
    END_STRUCT ;
    DataTimeFeedback : STRUCT
     StartTime : DINT ;
     StartEdge : BOOL ;
    END_STRUCT ;
    DataTimeActFault : STRUCT
     StartTime : DINT ;
     StartEdge : BOOL ;
    END_STRUCT ;
    DataTimeAutoAl : STRUCT
     StartTime : DINT ;
     StartEdge : BOOL ;
    END_STRUCT ;
    DataTimeRestart : STRUCT
     StartTime : DINT ;
     StartEdge : BOOL ;
    END_STRUCT ;
    DataTimeChgSF : STRUCT
     StartTime : DINT ;
     StartEdge : BOOL ;
    END_STRUCT ;
    DataTimeChgFS : STRUCT
     StartTime : DINT ;
     StartEdge : BOOL ;
    END_STRUCT ;
    DataTimeChgDirec : STRUCT
     StartTime : DINT ;
     StartEdge : BOOL ;
    END_STRUCT ;
    PCONF : STRUCT 	//// PCONF MOTOR3 - Instance 016
     Modeswitches : STRUCT
      M0_ConstantOut : BOOL ;	// Constant Output MST1 MST2 MSTO (1); Feedback depended Output Anst. (0)
      M1_AutoManLoc : BOOL ;	// AUTO/ MANUAL/ LOCAL (1); MANUAL/ LOCAL (0)
      M2_NoActFeedFault : BOOL ;	// No Action- and Non-Feedback fault(1),
      M3_NoStopIfFault : BOOL ;	// No Stop-Signal if Failure occurs (1)
      M4_RestrtAftBlack : BOOL ;	// Restart after Blackout (1)
      M5_ResetOSonly : BOOL ;	// Reset Alarm only with RESET from OS (1); RESET and START/STOP-Command (0)
      sw06 : BOOL ;
      M7_ChgSFviaStop : BOOL ;	// Change from Slow->Fast via STOP(1)
      M8_ChgFSviaStop : BOOL ;	// Change from Fast->Slow via STOP(1)
      M9_StopIfAutoFail : BOOL ;	// Direct Stop if Auto Failure (1)
      M10_ExtFaultNC : BOOL ;	// External Fault is NC (1)
      sw11 : BOOL ;
      sw12 : BOOL ;
      sw13 : BOOL ;
      sw14 : BOOL ;
      sw15 : BOOL ;	//
     END_STRUCT ;
     DlyTExtFault : TIME ;	// Setpoint external fault delay
     DlyTFeedback : TIME ;	// Setpoint feedback fault delay
     DlyTActFault : TIME ;	// Setpoint Action Fault delay
     DlyTAutoAl : TIME ;	// Setpoint auto alarm delay
     DlyTRestart : TIME ;	// Setpoint restart after blackout delay
     DlyTChgSF : TIME ;	// Setpoint Waiting Delay Slow->Fast
     DlyTChgFS : TIME ;	// Setpoint Waiting Delay Fast->Slow
     DlyTChgDirec : TIME ;	// Setpoint change direction
    END_STRUCT ;
   END_STRUCT ;
   MOTOR3_No017 : STRUCT
    System : WORD ;
    CmdOS : WORD ;
    MirrorCmdOS : WORD ;
    Test : WORD ;
    AlarmOS : WORD ;
    StatusOS : WORD ;
    SysStatusOS : WORD ;
    Status1 : WORD ;
    Status2 : WORD ;
    Status3 : BYTE ;
    InputEdges : BYTE ;
    AutoEdges : WORD ;
    DataTimeExtFault : STRUCT
     StartTime : DINT ;
     StartEdge : BOOL ;
    END_STRUCT ;
    DataTimeFeedback : STRUCT
     StartTime : DINT ;
     StartEdge : BOOL ;
    END_STRUCT ;
    DataTimeActFault : STRUCT
     StartTime : DINT ;
     StartEdge : BOOL ;
    END_STRUCT ;
    DataTimeAutoAl : STRUCT
     StartTime : DINT ;
     StartEdge : BOOL ;
    END_STRUCT ;
    DataTimeRestart : STRUCT
     StartTime : DINT ;
     StartEdge : BOOL ;
    END_STRUCT ;
    DataTimeChgSF : STRUCT
     StartTime : DINT ;
     StartEdge : BOOL ;
    END_STRUCT ;
    DataTimeChgFS : STRUCT
     StartTime : DINT ;
     StartEdge : BOOL ;
    END_STRUCT ;
    DataTimeChgDirec : STRUCT
     StartTime : DINT ;
     StartEdge : BOOL ;
    END_STRUCT ;
    PCONF : STRUCT 	//// PCONF MOTOR3 - Instance 017
     Modeswitches : STRUCT
      M0_ConstantOut : BOOL ;	// Constant Output MST1 MST2 MSTO (1); Feedback depended Output Anst. (0)
      M1_AutoManLoc : BOOL ;	// AUTO/ MANUAL/ LOCAL (1); MANUAL/ LOCAL (0)
      M2_NoActFeedFault : BOOL ;	// No Action- and Non-Feedback fault(1),
      M3_NoStopIfFault : BOOL ;	// No Stop-Signal if Failure occurs (1)
      M4_RestrtAftBlack : BOOL ;	// Restart after Blackout (1)
      M5_ResetOSonly : BOOL ;	// Reset Alarm only with RESET from OS (1); RESET and START/STOP-Command (0)
      sw06 : BOOL ;
      M7_ChgSFviaStop : BOOL ;	// Change from Slow->Fast via STOP(1)
      M8_ChgFSviaStop : BOOL ;	// Change from Fast->Slow via STOP(1)
      M9_StopIfAutoFail : BOOL ;	// Direct Stop if Auto Failure (1)
      M10_ExtFaultNC : BOOL ;	// External Fault is NC (1)
      sw11 : BOOL ;
      sw12 : BOOL ;
      sw13 : BOOL ;
      sw14 : BOOL ;
      sw15 : BOOL ;	//
     END_STRUCT ;
     DlyTExtFault : TIME ;	// Setpoint external fault delay
     DlyTFeedback : TIME ;	// Setpoint feedback fault delay
     DlyTActFault : TIME ;	// Setpoint Action Fault delay
     DlyTAutoAl : TIME ;	// Setpoint auto alarm delay
     DlyTRestart : TIME ;	// Setpoint restart after blackout delay
     DlyTChgSF : TIME ;	// Setpoint Waiting Delay Slow->Fast
     DlyTChgFS : TIME ;	// Setpoint Waiting Delay Fast->Slow
     DlyTChgDirec : TIME ;	// Setpoint change direction
    END_STRUCT ;
   END_STRUCT ;
   MOTOR3_No018 : STRUCT
    System : WORD ;
    CmdOS : WORD ;
    MirrorCmdOS : WORD ;
    Test : WORD ;
    AlarmOS : WORD ;
    StatusOS : WORD ;
    SysStatusOS : WORD ;
    Status1 : WORD ;
    Status2 : WORD ;
    Status3 : BYTE ;
    InputEdges : BYTE ;
    AutoEdges : WORD ;
    DataTimeExtFault : STRUCT
     StartTime : DINT ;
     StartEdge : BOOL ;
    END_STRUCT ;
    DataTimeFeedback : STRUCT
     StartTime : DINT ;
     StartEdge : BOOL ;
    END_STRUCT ;
    DataTimeActFault : STRUCT
     StartTime : DINT ;
     StartEdge : BOOL ;
    END_STRUCT ;
    DataTimeAutoAl : STRUCT
     StartTime : DINT ;
     StartEdge : BOOL ;
    END_STRUCT ;
    DataTimeRestart : STRUCT
     StartTime : DINT ;
     StartEdge : BOOL ;
    END_STRUCT ;
    DataTimeChgSF : STRUCT
     StartTime : DINT ;
     StartEdge : BOOL ;
    END_STRUCT ;
    DataTimeChgFS : STRUCT
     StartTime : DINT ;
     StartEdge : BOOL ;
    END_STRUCT ;
    DataTimeChgDirec : STRUCT
     StartTime : DINT ;
     StartEdge : BOOL ;
    END_STRUCT ;
    PCONF : STRUCT 	//// PCONF MOTOR3 - Instance 018
     Modeswitches : STRUCT
      M0_ConstantOut : BOOL ;	// Constant Output MST1 MST2 MSTO (1); Feedback depended Output Anst. (0)
      M1_AutoManLoc : BOOL ;	// AUTO/ MANUAL/ LOCAL (1); MANUAL/ LOCAL (0)
      M2_NoActFeedFault : BOOL ;	// No Action- and Non-Feedback fault(1),
      M3_NoStopIfFault : BOOL ;	// No Stop-Signal if Failure occurs (1)
      M4_RestrtAftBlack : BOOL ;	// Restart after Blackout (1)
      M5_ResetOSonly : BOOL ;	// Reset Alarm only with RESET from OS (1); RESET and START/STOP-Command (0)
      sw06 : BOOL ;
      M7_ChgSFviaStop : BOOL ;	// Change from Slow->Fast via STOP(1)
      M8_ChgFSviaStop : BOOL ;	// Change from Fast->Slow via STOP(1)
      M9_StopIfAutoFail : BOOL ;	// Direct Stop if Auto Failure (1)
      M10_ExtFaultNC : BOOL ;	// External Fault is NC (1)
      sw11 : BOOL ;
      sw12 : BOOL ;
      sw13 : BOOL ;
      sw14 : BOOL ;
      sw15 : BOOL ;	//
     END_STRUCT ;
     DlyTExtFault : TIME ;	// Setpoint external fault delay
     DlyTFeedback : TIME ;	// Setpoint feedback fault delay
     DlyTActFault : TIME ;	// Setpoint Action Fault delay
     DlyTAutoAl : TIME ;	// Setpoint auto alarm delay
     DlyTRestart : TIME ;	// Setpoint restart after blackout delay
     DlyTChgSF : TIME ;	// Setpoint Waiting Delay Slow->Fast
     DlyTChgFS : TIME ;	// Setpoint Waiting Delay Fast->Slow
     DlyTChgDirec : TIME ;	// Setpoint change direction
    END_STRUCT ;
   END_STRUCT ;
   MOTOR3_No019 : STRUCT
    System : WORD ;
    CmdOS : WORD ;
    MirrorCmdOS : WORD ;
    Test : WORD ;
    AlarmOS : WORD ;
    StatusOS : WORD ;
    SysStatusOS : WORD ;
    Status1 : WORD ;
    Status2 : WORD ;
    Status3 : BYTE ;
    InputEdges : BYTE ;
    AutoEdges : WORD ;
    DataTimeExtFault : STRUCT
     StartTime : DINT ;
     StartEdge : BOOL ;
    END_STRUCT ;
    DataTimeFeedback : STRUCT
     StartTime : DINT ;
     StartEdge : BOOL ;
    END_STRUCT ;
    DataTimeActFault : STRUCT
     StartTime : DINT ;
     StartEdge : BOOL ;
    END_STRUCT ;
    DataTimeAutoAl : STRUCT
     StartTime : DINT ;
     StartEdge : BOOL ;
    END_STRUCT ;
    DataTimeRestart : STRUCT
     StartTime : DINT ;
     StartEdge : BOOL ;
    END_STRUCT ;
    DataTimeChgSF : STRUCT
     StartTime : DINT ;
     StartEdge : BOOL ;
    END_STRUCT ;
    DataTimeChgFS : STRUCT
     StartTime : DINT ;
     StartEdge : BOOL ;
    END_STRUCT ;
    DataTimeChgDirec : STRUCT
     StartTime : DINT ;
     StartEdge : BOOL ;
    END_STRUCT ;
    PCONF : STRUCT 	//// PCONF MOTOR3 - Instance 019
     Modeswitches : STRUCT
      M0_ConstantOut : BOOL ;	// Constant Output MST1 MST2 MSTO (1); Feedback depended Output Anst. (0)
      M1_AutoManLoc : BOOL ;	// AUTO/ MANUAL/ LOCAL (1); MANUAL/ LOCAL (0)
      M2_NoActFeedFault : BOOL ;	// No Action- and Non-Feedback fault(1),
      M3_NoStopIfFault : BOOL ;	// No Stop-Signal if Failure occurs (1)
      M4_RestrtAftBlack : BOOL ;	// Restart after Blackout (1)
      M5_ResetOSonly : BOOL ;	// Reset Alarm only with RESET from OS (1); RESET and START/STOP-Command (0)
      sw06 : BOOL ;
      M7_ChgSFviaStop : BOOL ;	// Change from Slow->Fast via STOP(1)
      M8_ChgFSviaStop : BOOL ;	// Change from Fast->Slow via STOP(1)
      M9_StopIfAutoFail : BOOL ;	// Direct Stop if Auto Failure (1)
      M10_ExtFaultNC : BOOL ;	// External Fault is NC (1)
      sw11 : BOOL ;
      sw12 : BOOL ;
      sw13 : BOOL ;
      sw14 : BOOL ;
      sw15 : BOOL ;	//
     END_STRUCT ;
     DlyTExtFault : TIME ;	// Setpoint external fault delay
     DlyTFeedback : TIME ;	// Setpoint feedback fault delay
     DlyTActFault : TIME ;	// Setpoint Action Fault delay
     DlyTAutoAl : TIME ;	// Setpoint auto alarm delay
     DlyTRestart : TIME ;	// Setpoint restart after blackout delay
     DlyTChgSF : TIME ;	// Setpoint Waiting Delay Slow->Fast
     DlyTChgFS : TIME ;	// Setpoint Waiting Delay Fast->Slow
     DlyTChgDirec : TIME ;	// Setpoint change direction
    END_STRUCT ;
   END_STRUCT ;
   MOTOR3_No020 : STRUCT
    System : WORD ;
    CmdOS : WORD ;
    MirrorCmdOS : WORD ;
    Test : WORD ;
    AlarmOS : WORD ;
    StatusOS : WORD ;
    SysStatusOS : WORD ;
    Status1 : WORD ;
    Status2 : WORD ;
    Status3 : BYTE ;
    InputEdges : BYTE ;
    AutoEdges : WORD ;
    DataTimeExtFault : STRUCT
     StartTime : DINT ;
     StartEdge : BOOL ;
    END_STRUCT ;
    DataTimeFeedback : STRUCT
     StartTime : DINT ;
     StartEdge : BOOL ;
    END_STRUCT ;
    DataTimeActFault : STRUCT
     StartTime : DINT ;
     StartEdge : BOOL ;
    END_STRUCT ;
    DataTimeAutoAl : STRUCT
     StartTime : DINT ;
     StartEdge : BOOL ;
    END_STRUCT ;
    DataTimeRestart : STRUCT
     StartTime : DINT ;
     StartEdge : BOOL ;
    END_STRUCT ;
    DataTimeChgSF : STRUCT
     StartTime : DINT ;
     StartEdge : BOOL ;
    END_STRUCT ;
    DataTimeChgFS : STRUCT
     StartTime : DINT ;
     StartEdge : BOOL ;
    END_STRUCT ;
    DataTimeChgDirec : STRUCT
     StartTime : DINT ;
     StartEdge : BOOL ;
    END_STRUCT ;
    PCONF : STRUCT 	//// PCONF MOTOR3 - Instance 020
     Modeswitches : STRUCT
      M0_ConstantOut : BOOL ;	// Constant Output MST1 MST2 MSTO (1); Feedback depended Output Anst. (0)
      M1_AutoManLoc : BOOL ;	// AUTO/ MANUAL/ LOCAL (1); MANUAL/ LOCAL (0)
      M2_NoActFeedFault : BOOL ;	// No Action- and Non-Feedback fault(1),
      M3_NoStopIfFault : BOOL ;	// No Stop-Signal if Failure occurs (1)
      M4_RestrtAftBlack : BOOL ;	// Restart after Blackout (1)
      M5_ResetOSonly : BOOL ;	// Reset Alarm only with RESET from OS (1); RESET and START/STOP-Command (0)
      sw06 : BOOL ;
      M7_ChgSFviaStop : BOOL ;	// Change from Slow->Fast via STOP(1)
      M8_ChgFSviaStop : BOOL ;	// Change from Fast->Slow via STOP(1)
      M9_StopIfAutoFail : BOOL ;	// Direct Stop if Auto Failure (1)
      M10_ExtFaultNC : BOOL ;	// External Fault is NC (1)
      sw11 : BOOL ;
      sw12 : BOOL ;
      sw13 : BOOL ;
      sw14 : BOOL ;
      sw15 : BOOL ;	//
     END_STRUCT ;
     DlyTExtFault : TIME ;	// Setpoint external fault delay
     DlyTFeedback : TIME ;	// Setpoint feedback fault delay
     DlyTActFault : TIME ;	// Setpoint Action Fault delay
     DlyTAutoAl : TIME ;	// Setpoint auto alarm delay
     DlyTRestart : TIME ;	// Setpoint restart after blackout delay
     DlyTChgSF : TIME ;	// Setpoint Waiting Delay Slow->Fast
     DlyTChgFS : TIME ;	// Setpoint Waiting Delay Fast->Slow
     DlyTChgDirec : TIME ;	// Setpoint change direction
    END_STRUCT ;
   END_STRUCT ;
   MOTOR3_No021 : STRUCT
    System : WORD ;
    CmdOS : WORD ;
    MirrorCmdOS : WORD ;
    Test : WORD ;
    AlarmOS : WORD ;
    StatusOS : WORD ;
    SysStatusOS : WORD ;
    Status1 : WORD ;
    Status2 : WORD ;
    Status3 : BYTE ;
    InputEdges : BYTE ;
    AutoEdges : WORD ;
    DataTimeExtFault : STRUCT
     StartTime : DINT ;
     StartEdge : BOOL ;
    END_STRUCT ;
    DataTimeFeedback : STRUCT
     StartTime : DINT ;
     StartEdge : BOOL ;
    END_STRUCT ;
    DataTimeActFault : STRUCT
     StartTime : DINT ;
     StartEdge : BOOL ;
    END_STRUCT ;
    DataTimeAutoAl : STRUCT
     StartTime : DINT ;
     StartEdge : BOOL ;
    END_STRUCT ;
    DataTimeRestart : STRUCT
     StartTime : DINT ;
     StartEdge : BOOL ;
    END_STRUCT ;
    DataTimeChgSF : STRUCT
     StartTime : DINT ;
     StartEdge : BOOL ;
    END_STRUCT ;
    DataTimeChgFS : STRUCT
     StartTime : DINT ;
     StartEdge : BOOL ;
    END_STRUCT ;
    DataTimeChgDirec : STRUCT
     StartTime : DINT ;
     StartEdge : BOOL ;
    END_STRUCT ;
    PCONF : STRUCT 	//// PCONF MOTOR3 - Instance 021
     Modeswitches : STRUCT
      M0_ConstantOut : BOOL ;	// Constant Output MST1 MST2 MSTO (1); Feedback depended Output Anst. (0)
      M1_AutoManLoc : BOOL ;	// AUTO/ MANUAL/ LOCAL (1); MANUAL/ LOCAL (0)
      M2_NoActFeedFault : BOOL ;	// No Action- and Non-Feedback fault(1),
      M3_NoStopIfFault : BOOL ;	// No Stop-Signal if Failure occurs (1)
      M4_RestrtAftBlack : BOOL ;	// Restart after Blackout (1)
      M5_ResetOSonly : BOOL ;	// Reset Alarm only with RESET from OS (1); RESET and START/STOP-Command (0)
      sw06 : BOOL ;
      M7_ChgSFviaStop : BOOL ;	// Change from Slow->Fast via STOP(1)
      M8_ChgFSviaStop : BOOL ;	// Change from Fast->Slow via STOP(1)
      M9_StopIfAutoFail : BOOL ;	// Direct Stop if Auto Failure (1)
      M10_ExtFaultNC : BOOL ;	// External Fault is NC (1)
      sw11 : BOOL ;
      sw12 : BOOL ;
      sw13 : BOOL ;
      sw14 : BOOL ;
      sw15 : BOOL ;	//
     END_STRUCT ;
     DlyTExtFault : TIME ;	// Setpoint external fault delay
     DlyTFeedback : TIME ;	// Setpoint feedback fault delay
     DlyTActFault : TIME ;	// Setpoint Action Fault delay
     DlyTAutoAl : TIME ;	// Setpoint auto alarm delay
     DlyTRestart : TIME ;	// Setpoint restart after blackout delay
     DlyTChgSF : TIME ;	// Setpoint Waiting Delay Slow->Fast
     DlyTChgFS : TIME ;	// Setpoint Waiting Delay Fast->Slow
     DlyTChgDirec : TIME ;	// Setpoint change direction
    END_STRUCT ;
   END_STRUCT ;
   MOTOR3_No022 : STRUCT
    System : WORD ;
    CmdOS : WORD ;
    MirrorCmdOS : WORD ;
    Test : WORD ;
    AlarmOS : WORD ;
    StatusOS : WORD ;
    SysStatusOS : WORD ;
    Status1 : WORD ;
    Status2 : WORD ;
    Status3 : BYTE ;
    InputEdges : BYTE ;
    AutoEdges : WORD ;
    DataTimeExtFault : STRUCT
     StartTime : DINT ;
     StartEdge : BOOL ;
    END_STRUCT ;
    DataTimeFeedback : STRUCT
     StartTime : DINT ;
     StartEdge : BOOL ;
    END_STRUCT ;
    DataTimeActFault : STRUCT
     StartTime : DINT ;
     StartEdge : BOOL ;
    END_STRUCT ;
    DataTimeAutoAl : STRUCT
     StartTime : DINT ;
     StartEdge : BOOL ;
    END_STRUCT ;
    DataTimeRestart : STRUCT
     StartTime : DINT ;
     StartEdge : BOOL ;
    END_STRUCT ;
    DataTimeChgSF : STRUCT
     StartTime : DINT ;
     StartEdge : BOOL ;
    END_STRUCT ;
    DataTimeChgFS : STRUCT
     StartTime : DINT ;
     StartEdge : BOOL ;
    END_STRUCT ;
    DataTimeChgDirec : STRUCT
     StartTime : DINT ;
     StartEdge : BOOL ;
    END_STRUCT ;
    PCONF : STRUCT 	//// PCONF MOTOR3 - Instance 022
     Modeswitches : STRUCT
      M0_ConstantOut : BOOL ;	// Constant Output MST1 MST2 MSTO (1); Feedback depended Output Anst. (0)
      M1_AutoManLoc : BOOL ;	// AUTO/ MANUAL/ LOCAL (1); MANUAL/ LOCAL (0)
      M2_NoActFeedFault : BOOL ;	// No Action- and Non-Feedback fault(1),
      M3_NoStopIfFault : BOOL ;	// No Stop-Signal if Failure occurs (1)
      M4_RestrtAftBlack : BOOL ;	// Restart after Blackout (1)
      M5_ResetOSonly : BOOL ;	// Reset Alarm only with RESET from OS (1); RESET and START/STOP-Command (0)
      sw06 : BOOL ;
      M7_ChgSFviaStop : BOOL ;	// Change from Slow->Fast via STOP(1)
      M8_ChgFSviaStop : BOOL ;	// Change from Fast->Slow via STOP(1)
      M9_StopIfAutoFail : BOOL ;	// Direct Stop if Auto Failure (1)
      M10_ExtFaultNC : BOOL ;	// External Fault is NC (1)
      sw11 : BOOL ;
      sw12 : BOOL ;
      sw13 : BOOL ;
      sw14 : BOOL ;
      sw15 : BOOL ;	//
     END_STRUCT ;
     DlyTExtFault : TIME ;	// Setpoint external fault delay
     DlyTFeedback : TIME ;	// Setpoint feedback fault delay
     DlyTActFault : TIME ;	// Setpoint Action Fault delay
     DlyTAutoAl : TIME ;	// Setpoint auto alarm delay
     DlyTRestart : TIME ;	// Setpoint restart after blackout delay
     DlyTChgSF : TIME ;	// Setpoint Waiting Delay Slow->Fast
     DlyTChgFS : TIME ;	// Setpoint Waiting Delay Fast->Slow
     DlyTChgDirec : TIME ;	// Setpoint change direction
    END_STRUCT ;
   END_STRUCT ;
   MOTOR3_No023 : STRUCT
    System : WORD ;
    CmdOS : WORD ;
    MirrorCmdOS : WORD ;
    Test : WORD ;
    AlarmOS : WORD ;
    StatusOS : WORD ;
    SysStatusOS : WORD ;
    Status1 : WORD ;
    Status2 : WORD ;
    Status3 : BYTE ;
    InputEdges : BYTE ;
    AutoEdges : WORD ;
    DataTimeExtFault : STRUCT
     StartTime : DINT ;
     StartEdge : BOOL ;
    END_STRUCT ;
    DataTimeFeedback : STRUCT
     StartTime : DINT ;
     StartEdge : BOOL ;
    END_STRUCT ;
    DataTimeActFault : STRUCT
     StartTime : DINT ;
     StartEdge : BOOL ;
    END_STRUCT ;
    DataTimeAutoAl : STRUCT
     StartTime : DINT ;
     StartEdge : BOOL ;
    END_STRUCT ;
    DataTimeRestart : STRUCT
     StartTime : DINT ;
     StartEdge : BOOL ;
    END_STRUCT ;
    DataTimeChgSF : STRUCT
     StartTime : DINT ;
     StartEdge : BOOL ;
    END_STRUCT ;
    DataTimeChgFS : STRUCT
     StartTime : DINT ;
     StartEdge : BOOL ;
    END_STRUCT ;
    DataTimeChgDirec : STRUCT
     StartTime : DINT ;
     StartEdge : BOOL ;
    END_STRUCT ;
    PCONF : STRUCT 	//// PCONF MOTOR3 - Instance 023
     Modeswitches : STRUCT
      M0_ConstantOut : BOOL ;	// Constant Output MST1 MST2 MSTO (1); Feedback depended Output Anst. (0)
      M1_AutoManLoc : BOOL ;	// AUTO/ MANUAL/ LOCAL (1); MANUAL/ LOCAL (0)
      M2_NoActFeedFault : BOOL ;	// No Action- and Non-Feedback fault(1),
      M3_NoStopIfFault : BOOL ;	// No Stop-Signal if Failure occurs (1)
      M4_RestrtAftBlack : BOOL ;	// Restart after Blackout (1)
      M5_ResetOSonly : BOOL ;	// Reset Alarm only with RESET from OS (1); RESET and START/STOP-Command (0)
      sw06 : BOOL ;
      M7_ChgSFviaStop : BOOL ;	// Change from Slow->Fast via STOP(1)
      M8_ChgFSviaStop : BOOL ;	// Change from Fast->Slow via STOP(1)
      M9_StopIfAutoFail : BOOL ;	// Direct Stop if Auto Failure (1)
      M10_ExtFaultNC : BOOL ;	// External Fault is NC (1)
      sw11 : BOOL ;
      sw12 : BOOL ;
      sw13 : BOOL ;
      sw14 : BOOL ;
      sw15 : BOOL ;	//
     END_STRUCT ;
     DlyTExtFault : TIME ;	// Setpoint external fault delay
     DlyTFeedback : TIME ;	// Setpoint feedback fault delay
     DlyTActFault : TIME ;	// Setpoint Action Fault delay
     DlyTAutoAl : TIME ;	// Setpoint auto alarm delay
     DlyTRestart : TIME ;	// Setpoint restart after blackout delay
     DlyTChgSF : TIME ;	// Setpoint Waiting Delay Slow->Fast
     DlyTChgFS : TIME ;	// Setpoint Waiting Delay Fast->Slow
     DlyTChgDirec : TIME ;	// Setpoint change direction
    END_STRUCT ;
   END_STRUCT ;
   MOTOR3_No024 : STRUCT
    System : WORD ;
    CmdOS : WORD ;
    MirrorCmdOS : WORD ;
    Test : WORD ;
    AlarmOS : WORD ;
    StatusOS : WORD ;
    SysStatusOS : WORD ;
    Status1 : WORD ;
    Status2 : WORD ;
    Status3 : BYTE ;
    InputEdges : BYTE ;
    AutoEdges : WORD ;
    DataTimeExtFault : STRUCT
     StartTime : DINT ;
     StartEdge : BOOL ;
    END_STRUCT ;
    DataTimeFeedback : STRUCT
     StartTime : DINT ;
     StartEdge : BOOL ;
    END_STRUCT ;
    DataTimeActFault : STRUCT
     StartTime : DINT ;
     StartEdge : BOOL ;
    END_STRUCT ;
    DataTimeAutoAl : STRUCT
     StartTime : DINT ;
     StartEdge : BOOL ;
    END_STRUCT ;
    DataTimeRestart : STRUCT
     StartTime : DINT ;
     StartEdge : BOOL ;
    END_STRUCT ;
    DataTimeChgSF : STRUCT
     StartTime : DINT ;
     StartEdge : BOOL ;
    END_STRUCT ;
    DataTimeChgFS : STRUCT
     StartTime : DINT ;
     StartEdge : BOOL ;
    END_STRUCT ;
    DataTimeChgDirec : STRUCT
     StartTime : DINT ;
     StartEdge : BOOL ;
    END_STRUCT ;
    PCONF : STRUCT 	//// PCONF MOTOR3 - Instance 024
     Modeswitches : STRUCT
      M0_ConstantOut : BOOL ;	// Constant Output MST1 MST2 MSTO (1); Feedback depended Output Anst. (0)
      M1_AutoManLoc : BOOL ;	// AUTO/ MANUAL/ LOCAL (1); MANUAL/ LOCAL (0)
      M2_NoActFeedFault : BOOL ;	// No Action- and Non-Feedback fault(1),
      M3_NoStopIfFault : BOOL ;	// No Stop-Signal if Failure occurs (1)
      M4_RestrtAftBlack : BOOL ;	// Restart after Blackout (1)
      M5_ResetOSonly : BOOL ;	// Reset Alarm only with RESET from OS (1); RESET and START/STOP-Command (0)
      sw06 : BOOL ;
      M7_ChgSFviaStop : BOOL ;	// Change from Slow->Fast via STOP(1)
      M8_ChgFSviaStop : BOOL ;	// Change from Fast->Slow via STOP(1)
      M9_StopIfAutoFail : BOOL ;	// Direct Stop if Auto Failure (1)
      M10_ExtFaultNC : BOOL ;	// External Fault is NC (1)
      sw11 : BOOL ;
      sw12 : BOOL ;
      sw13 : BOOL ;
      sw14 : BOOL ;
      sw15 : BOOL ;	//
     END_STRUCT ;
     DlyTExtFault : TIME ;	// Setpoint external fault delay
     DlyTFeedback : TIME ;	// Setpoint feedback fault delay
     DlyTActFault : TIME ;	// Setpoint Action Fault delay
     DlyTAutoAl : TIME ;	// Setpoint auto alarm delay
     DlyTRestart : TIME ;	// Setpoint restart after blackout delay
     DlyTChgSF : TIME ;	// Setpoint Waiting Delay Slow->Fast
     DlyTChgFS : TIME ;	// Setpoint Waiting Delay Fast->Slow
     DlyTChgDirec : TIME ;	// Setpoint change direction
    END_STRUCT ;
   END_STRUCT ;
   MOTOR3_No025 : STRUCT
    System : WORD ;
    CmdOS : WORD ;
    MirrorCmdOS : WORD ;
    Test : WORD ;
    AlarmOS : WORD ;
    StatusOS : WORD ;
    SysStatusOS : WORD ;
    Status1 : WORD ;
    Status2 : WORD ;
    Status3 : BYTE ;
    InputEdges : BYTE ;
    AutoEdges : WORD ;
    DataTimeExtFault : STRUCT
     StartTime : DINT ;
     StartEdge : BOOL ;
    END_STRUCT ;
    DataTimeFeedback : STRUCT
     StartTime : DINT ;
     StartEdge : BOOL ;
    END_STRUCT ;
    DataTimeActFault : STRUCT
     StartTime : DINT ;
     StartEdge : BOOL ;
    END_STRUCT ;
    DataTimeAutoAl : STRUCT
     StartTime : DINT ;
     StartEdge : BOOL ;
    END_STRUCT ;
    DataTimeRestart : STRUCT
     StartTime : DINT ;
     StartEdge : BOOL ;
    END_STRUCT ;
    DataTimeChgSF : STRUCT
     StartTime : DINT ;
     StartEdge : BOOL ;
    END_STRUCT ;
    DataTimeChgFS : STRUCT
     StartTime : DINT ;
     StartEdge : BOOL ;
    END_STRUCT ;
    DataTimeChgDirec : STRUCT
     StartTime : DINT ;
     StartEdge : BOOL ;
    END_STRUCT ;
    PCONF : STRUCT 	//// PCONF MOTOR3 - Instance 025
     Modeswitches : STRUCT
      M0_ConstantOut : BOOL ;	// Constant Output MST1 MST2 MSTO (1); Feedback depended Output Anst. (0)
      M1_AutoManLoc : BOOL ;	// AUTO/ MANUAL/ LOCAL (1); MANUAL/ LOCAL (0)
      M2_NoActFeedFault : BOOL ;	// No Action- and Non-Feedback fault(1),
      M3_NoStopIfFault : BOOL ;	// No Stop-Signal if Failure occurs (1)
      M4_RestrtAftBlack : BOOL ;	// Restart after Blackout (1)
      M5_ResetOSonly : BOOL ;	// Reset Alarm only with RESET from OS (1); RESET and START/STOP-Command (0)
      sw06 : BOOL ;
      M7_ChgSFviaStop : BOOL ;	// Change from Slow->Fast via STOP(1)
      M8_ChgFSviaStop : BOOL ;	// Change from Fast->Slow via STOP(1)
      M9_StopIfAutoFail : BOOL ;	// Direct Stop if Auto Failure (1)
      M10_ExtFaultNC : BOOL ;	// External Fault is NC (1)
      sw11 : BOOL ;
      sw12 : BOOL ;
      sw13 : BOOL ;
      sw14 : BOOL ;
      sw15 : BOOL ;	//
     END_STRUCT ;
     DlyTExtFault : TIME ;	// Setpoint external fault delay
     DlyTFeedback : TIME ;	// Setpoint feedback fault delay
     DlyTActFault : TIME ;	// Setpoint Action Fault delay
     DlyTAutoAl : TIME ;	// Setpoint auto alarm delay
     DlyTRestart : TIME ;	// Setpoint restart after blackout delay
     DlyTChgSF : TIME ;	// Setpoint Waiting Delay Slow->Fast
     DlyTChgFS : TIME ;	// Setpoint Waiting Delay Fast->Slow
     DlyTChgDirec : TIME ;	// Setpoint change direction
    END_STRUCT ;
   END_STRUCT ;
  END_STRUCT ;
BEGIN
   MOTOR3_No001.System := W#16#0;
   MOTOR3_No001.CmdOS := W#16#0;
   MOTOR3_No001.MirrorCmdOS := W#16#0;
   MOTOR3_No001.Test := W#16#0;
   MOTOR3_No001.AlarmOS := W#16#0;
   MOTOR3_No001.StatusOS := W#16#0;
   MOTOR3_No001.SysStatusOS := W#16#0;
   MOTOR3_No001.Status1 := W#16#0;
   MOTOR3_No001.Status2 := W#16#0;
   MOTOR3_No001.Status3 := B#16#0;
   MOTOR3_No001.InputEdges := B#16#0;
   MOTOR3_No001.AutoEdges := W#16#0;
   MOTOR3_No001.DataTimeExtFault.StartTime := L#0;
   MOTOR3_No001.DataTimeExtFault.StartEdge := FALSE;
   MOTOR3_No001.DataTimeFeedback.StartTime := L#0;
   MOTOR3_No001.DataTimeFeedback.StartEdge := FALSE;
   MOTOR3_No001.DataTimeActFault.StartTime := L#0;
   MOTOR3_No001.DataTimeActFault.StartEdge := FALSE;
   MOTOR3_No001.DataTimeAutoAl.StartTime := L#0;
   MOTOR3_No001.DataTimeAutoAl.StartEdge := FALSE;
   MOTOR3_No001.DataTimeRestart.StartTime := L#0;
   MOTOR3_No001.DataTimeRestart.StartEdge := FALSE;
   MOTOR3_No001.DataTimeChgSF.StartTime := L#0;
   MOTOR3_No001.DataTimeChgSF.StartEdge := FALSE;
   MOTOR3_No001.DataTimeChgFS.StartTime := L#0;
   MOTOR3_No001.DataTimeChgFS.StartEdge := FALSE;
   MOTOR3_No001.DataTimeChgDirec.StartTime := L#0;
   MOTOR3_No001.DataTimeChgDirec.StartEdge := FALSE;
   MOTOR3_No001.PCONF.Modeswitches.M0_ConstantOut := TRUE;
   MOTOR3_No001.PCONF.Modeswitches.M1_AutoManLoc := TRUE;
   MOTOR3_No001.PCONF.Modeswitches.M2_NoActFeedFault := FALSE;
   MOTOR3_No001.PCONF.Modeswitches.M3_NoStopIfFault := TRUE;
   MOTOR3_No001.PCONF.Modeswitches.M4_RestrtAftBlack := TRUE;
   MOTOR3_No001.PCONF.Modeswitches.M5_ResetOSonly := TRUE;
   MOTOR3_No001.PCONF.Modeswitches.sw06 := FALSE;
   MOTOR3_No001.PCONF.Modeswitches.M7_ChgSFviaStop := FALSE;
   MOTOR3_No001.PCONF.Modeswitches.M8_ChgFSviaStop := FALSE;
   MOTOR3_No001.PCONF.Modeswitches.M9_StopIfAutoFail := FALSE;
   MOTOR3_No001.PCONF.Modeswitches.M10_ExtFaultNC := FALSE;
   MOTOR3_No001.PCONF.Modeswitches.sw11 := FALSE;
   MOTOR3_No001.PCONF.Modeswitches.sw12 := FALSE;
   MOTOR3_No001.PCONF.Modeswitches.sw13 := FALSE;
   MOTOR3_No001.PCONF.Modeswitches.sw14 := FALSE;
   MOTOR3_No001.PCONF.Modeswitches.sw15 := FALSE;
   MOTOR3_No001.PCONF.DlyTExtFault := T#1S;
   MOTOR3_No001.PCONF.DlyTFeedback := T#1S;
   MOTOR3_No001.PCONF.DlyTActFault := T#5S;
   MOTOR3_No001.PCONF.DlyTAutoAl := T#1S;
   MOTOR3_No001.PCONF.DlyTRestart := T#40S;
   MOTOR3_No001.PCONF.DlyTChgSF := T#1S;
   MOTOR3_No001.PCONF.DlyTChgFS := T#2S;
   MOTOR3_No001.PCONF.DlyTChgDirec := T#4S;
   MOTOR3_No002.System := W#16#0;
   MOTOR3_No002.CmdOS := W#16#0;
   MOTOR3_No002.MirrorCmdOS := W#16#0;
   MOTOR3_No002.Test := W#16#0;
   MOTOR3_No002.AlarmOS := W#16#0;
   MOTOR3_No002.StatusOS := W#16#0;
   MOTOR3_No002.SysStatusOS := W#16#0;
   MOTOR3_No002.Status1 := W#16#0;
   MOTOR3_No002.Status2 := W#16#0;
   MOTOR3_No002.Status3 := B#16#0;
   MOTOR3_No002.InputEdges := B#16#0;
   MOTOR3_No002.AutoEdges := W#16#0;
   MOTOR3_No002.DataTimeExtFault.StartTime := L#0;
   MOTOR3_No002.DataTimeExtFault.StartEdge := FALSE;
   MOTOR3_No002.DataTimeFeedback.StartTime := L#0;
   MOTOR3_No002.DataTimeFeedback.StartEdge := FALSE;
   MOTOR3_No002.DataTimeActFault.StartTime := L#0;
   MOTOR3_No002.DataTimeActFault.StartEdge := FALSE;
   MOTOR3_No002.DataTimeAutoAl.StartTime := L#0;
   MOTOR3_No002.DataTimeAutoAl.StartEdge := FALSE;
   MOTOR3_No002.DataTimeRestart.StartTime := L#0;
   MOTOR3_No002.DataTimeRestart.StartEdge := FALSE;
   MOTOR3_No002.DataTimeChgSF.StartTime := L#0;
   MOTOR3_No002.DataTimeChgSF.StartEdge := FALSE;
   MOTOR3_No002.DataTimeChgFS.StartTime := L#0;
   MOTOR3_No002.DataTimeChgFS.StartEdge := FALSE;
   MOTOR3_No002.DataTimeChgDirec.StartTime := L#0;
   MOTOR3_No002.DataTimeChgDirec.StartEdge := FALSE;
   MOTOR3_No002.PCONF.Modeswitches.M0_ConstantOut := FALSE;
   MOTOR3_No002.PCONF.Modeswitches.M1_AutoManLoc := FALSE;
   MOTOR3_No002.PCONF.Modeswitches.M2_NoActFeedFault := FALSE;
   MOTOR3_No002.PCONF.Modeswitches.M3_NoStopIfFault := FALSE;
   MOTOR3_No002.PCONF.Modeswitches.M4_RestrtAftBlack := FALSE;
   MOTOR3_No002.PCONF.Modeswitches.M5_ResetOSonly := FALSE;
   MOTOR3_No002.PCONF.Modeswitches.sw06 := FALSE;
   MOTOR3_No002.PCONF.Modeswitches.M7_ChgSFviaStop := FALSE;
   MOTOR3_No002.PCONF.Modeswitches.M8_ChgFSviaStop := FALSE;
   MOTOR3_No002.PCONF.Modeswitches.M9_StopIfAutoFail := FALSE;
   MOTOR3_No002.PCONF.Modeswitches.M10_ExtFaultNC := FALSE;
   MOTOR3_No002.PCONF.Modeswitches.sw11 := FALSE;
   MOTOR3_No002.PCONF.Modeswitches.sw12 := FALSE;
   MOTOR3_No002.PCONF.Modeswitches.sw13 := FALSE;
   MOTOR3_No002.PCONF.Modeswitches.sw14 := FALSE;
   MOTOR3_No002.PCONF.Modeswitches.sw15 := FALSE;
   MOTOR3_No002.PCONF.DlyTExtFault := T#0MS;
   MOTOR3_No002.PCONF.DlyTFeedback := T#0MS;
   MOTOR3_No002.PCONF.DlyTActFault := T#0MS;
   MOTOR3_No002.PCONF.DlyTAutoAl := T#0MS;
   MOTOR3_No002.PCONF.DlyTRestart := T#0MS;
   MOTOR3_No002.PCONF.DlyTChgSF := T#0MS;
   MOTOR3_No002.PCONF.DlyTChgFS := T#0MS;
   MOTOR3_No002.PCONF.DlyTChgDirec := T#0MS;
   MOTOR3_No003.System := W#16#0;
   MOTOR3_No003.CmdOS := W#16#0;
   MOTOR3_No003.MirrorCmdOS := W#16#0;
   MOTOR3_No003.Test := W#16#0;
   MOTOR3_No003.AlarmOS := W#16#0;
   MOTOR3_No003.StatusOS := W#16#0;
   MOTOR3_No003.SysStatusOS := W#16#0;
   MOTOR3_No003.Status1 := W#16#0;
   MOTOR3_No003.Status2 := W#16#0;
   MOTOR3_No003.Status3 := B#16#0;
   MOTOR3_No003.InputEdges := B#16#0;
   MOTOR3_No003.AutoEdges := W#16#0;
   MOTOR3_No003.DataTimeExtFault.StartTime := L#0;
   MOTOR3_No003.DataTimeExtFault.StartEdge := FALSE;
   MOTOR3_No003.DataTimeFeedback.StartTime := L#0;
   MOTOR3_No003.DataTimeFeedback.StartEdge := FALSE;
   MOTOR3_No003.DataTimeActFault.StartTime := L#0;
   MOTOR3_No003.DataTimeActFault.StartEdge := FALSE;
   MOTOR3_No003.DataTimeAutoAl.StartTime := L#0;
   MOTOR3_No003.DataTimeAutoAl.StartEdge := FALSE;
   MOTOR3_No003.DataTimeRestart.StartTime := L#0;
   MOTOR3_No003.DataTimeRestart.StartEdge := FALSE;
   MOTOR3_No003.DataTimeChgSF.StartTime := L#0;
   MOTOR3_No003.DataTimeChgSF.StartEdge := FALSE;
   MOTOR3_No003.DataTimeChgFS.StartTime := L#0;
   MOTOR3_No003.DataTimeChgFS.StartEdge := FALSE;
   MOTOR3_No003.DataTimeChgDirec.StartTime := L#0;
   MOTOR3_No003.DataTimeChgDirec.StartEdge := FALSE;
   MOTOR3_No003.PCONF.Modeswitches.M0_ConstantOut := FALSE;
   MOTOR3_No003.PCONF.Modeswitches.M1_AutoManLoc := FALSE;
   MOTOR3_No003.PCONF.Modeswitches.M2_NoActFeedFault := FALSE;
   MOTOR3_No003.PCONF.Modeswitches.M3_NoStopIfFault := FALSE;
   MOTOR3_No003.PCONF.Modeswitches.M4_RestrtAftBlack := FALSE;
   MOTOR3_No003.PCONF.Modeswitches.M5_ResetOSonly := FALSE;
   MOTOR3_No003.PCONF.Modeswitches.sw06 := FALSE;
   MOTOR3_No003.PCONF.Modeswitches.M7_ChgSFviaStop := FALSE;
   MOTOR3_No003.PCONF.Modeswitches.M8_ChgFSviaStop := FALSE;
   MOTOR3_No003.PCONF.Modeswitches.M9_StopIfAutoFail := FALSE;
   MOTOR3_No003.PCONF.Modeswitches.M10_ExtFaultNC := FALSE;
   MOTOR3_No003.PCONF.Modeswitches.sw11 := FALSE;
   MOTOR3_No003.PCONF.Modeswitches.sw12 := FALSE;
   MOTOR3_No003.PCONF.Modeswitches.sw13 := FALSE;
   MOTOR3_No003.PCONF.Modeswitches.sw14 := FALSE;
   MOTOR3_No003.PCONF.Modeswitches.sw15 := FALSE;
   MOTOR3_No003.PCONF.DlyTExtFault := T#0MS;
   MOTOR3_No003.PCONF.DlyTFeedback := T#0MS;
   MOTOR3_No003.PCONF.DlyTActFault := T#0MS;
   MOTOR3_No003.PCONF.DlyTAutoAl := T#0MS;
   MOTOR3_No003.PCONF.DlyTRestart := T#0MS;
   MOTOR3_No003.PCONF.DlyTChgSF := T#0MS;
   MOTOR3_No003.PCONF.DlyTChgFS := T#0MS;
   MOTOR3_No003.PCONF.DlyTChgDirec := T#0MS;
   MOTOR3_No004.System := W#16#0;
   MOTOR3_No004.CmdOS := W#16#0;
   MOTOR3_No004.MirrorCmdOS := W#16#0;
   MOTOR3_No004.Test := W#16#0;
   MOTOR3_No004.AlarmOS := W#16#0;
   MOTOR3_No004.StatusOS := W#16#0;
   MOTOR3_No004.SysStatusOS := W#16#0;
   MOTOR3_No004.Status1 := W#16#0;
   MOTOR3_No004.Status2 := W#16#0;
   MOTOR3_No004.Status3 := B#16#0;
   MOTOR3_No004.InputEdges := B#16#0;
   MOTOR3_No004.AutoEdges := W#16#0;
   MOTOR3_No004.DataTimeExtFault.StartTime := L#0;
   MOTOR3_No004.DataTimeExtFault.StartEdge := FALSE;
   MOTOR3_No004.DataTimeFeedback.StartTime := L#0;
   MOTOR3_No004.DataTimeFeedback.StartEdge := FALSE;
   MOTOR3_No004.DataTimeActFault.StartTime := L#0;
   MOTOR3_No004.DataTimeActFault.StartEdge := FALSE;
   MOTOR3_No004.DataTimeAutoAl.StartTime := L#0;
   MOTOR3_No004.DataTimeAutoAl.StartEdge := FALSE;
   MOTOR3_No004.DataTimeRestart.StartTime := L#0;
   MOTOR3_No004.DataTimeRestart.StartEdge := FALSE;
   MOTOR3_No004.DataTimeChgSF.StartTime := L#0;
   MOTOR3_No004.DataTimeChgSF.StartEdge := FALSE;
   MOTOR3_No004.DataTimeChgFS.StartTime := L#0;
   MOTOR3_No004.DataTimeChgFS.StartEdge := FALSE;
   MOTOR3_No004.DataTimeChgDirec.StartTime := L#0;
   MOTOR3_No004.DataTimeChgDirec.StartEdge := FALSE;
   MOTOR3_No004.PCONF.Modeswitches.M0_ConstantOut := FALSE;
   MOTOR3_No004.PCONF.Modeswitches.M1_AutoManLoc := FALSE;
   MOTOR3_No004.PCONF.Modeswitches.M2_NoActFeedFault := FALSE;
   MOTOR3_No004.PCONF.Modeswitches.M3_NoStopIfFault := FALSE;
   MOTOR3_No004.PCONF.Modeswitches.M4_RestrtAftBlack := FALSE;
   MOTOR3_No004.PCONF.Modeswitches.M5_ResetOSonly := FALSE;
   MOTOR3_No004.PCONF.Modeswitches.sw06 := FALSE;
   MOTOR3_No004.PCONF.Modeswitches.M7_ChgSFviaStop := FALSE;
   MOTOR3_No004.PCONF.Modeswitches.M8_ChgFSviaStop := FALSE;
   MOTOR3_No004.PCONF.Modeswitches.M9_StopIfAutoFail := FALSE;
   MOTOR3_No004.PCONF.Modeswitches.M10_ExtFaultNC := FALSE;
   MOTOR3_No004.PCONF.Modeswitches.sw11 := FALSE;
   MOTOR3_No004.PCONF.Modeswitches.sw12 := FALSE;
   MOTOR3_No004.PCONF.Modeswitches.sw13 := FALSE;
   MOTOR3_No004.PCONF.Modeswitches.sw14 := FALSE;
   MOTOR3_No004.PCONF.Modeswitches.sw15 := FALSE;
   MOTOR3_No004.PCONF.DlyTExtFault := T#0MS;
   MOTOR3_No004.PCONF.DlyTFeedback := T#0MS;
   MOTOR3_No004.PCONF.DlyTActFault := T#0MS;
   MOTOR3_No004.PCONF.DlyTAutoAl := T#0MS;
   MOTOR3_No004.PCONF.DlyTRestart := T#0MS;
   MOTOR3_No004.PCONF.DlyTChgSF := T#0MS;
   MOTOR3_No004.PCONF.DlyTChgFS := T#0MS;
   MOTOR3_No004.PCONF.DlyTChgDirec := T#0MS;
   MOTOR3_No005.System := W#16#0;
   MOTOR3_No005.CmdOS := W#16#0;
   MOTOR3_No005.MirrorCmdOS := W#16#0;
   MOTOR3_No005.Test := W#16#0;
   MOTOR3_No005.AlarmOS := W#16#0;
   MOTOR3_No005.StatusOS := W#16#0;
   MOTOR3_No005.SysStatusOS := W#16#0;
   MOTOR3_No005.Status1 := W#16#0;
   MOTOR3_No005.Status2 := W#16#0;
   MOTOR3_No005.Status3 := B#16#0;
   MOTOR3_No005.InputEdges := B#16#0;
   MOTOR3_No005.AutoEdges := W#16#0;
   MOTOR3_No005.DataTimeExtFault.StartTime := L#0;
   MOTOR3_No005.DataTimeExtFault.StartEdge := FALSE;
   MOTOR3_No005.DataTimeFeedback.StartTime := L#0;
   MOTOR3_No005.DataTimeFeedback.StartEdge := FALSE;
   MOTOR3_No005.DataTimeActFault.StartTime := L#0;
   MOTOR3_No005.DataTimeActFault.StartEdge := FALSE;
   MOTOR3_No005.DataTimeAutoAl.StartTime := L#0;
   MOTOR3_No005.DataTimeAutoAl.StartEdge := FALSE;
   MOTOR3_No005.DataTimeRestart.StartTime := L#0;
   MOTOR3_No005.DataTimeRestart.StartEdge := FALSE;
   MOTOR3_No005.DataTimeChgSF.StartTime := L#0;
   MOTOR3_No005.DataTimeChgSF.StartEdge := FALSE;
   MOTOR3_No005.DataTimeChgFS.StartTime := L#0;
   MOTOR3_No005.DataTimeChgFS.StartEdge := FALSE;
   MOTOR3_No005.DataTimeChgDirec.StartTime := L#0;
   MOTOR3_No005.DataTimeChgDirec.StartEdge := FALSE;
   MOTOR3_No005.PCONF.Modeswitches.M0_ConstantOut := FALSE;
   MOTOR3_No005.PCONF.Modeswitches.M1_AutoManLoc := FALSE;
   MOTOR3_No005.PCONF.Modeswitches.M2_NoActFeedFault := FALSE;
   MOTOR3_No005.PCONF.Modeswitches.M3_NoStopIfFault := FALSE;
   MOTOR3_No005.PCONF.Modeswitches.M4_RestrtAftBlack := FALSE;
   MOTOR3_No005.PCONF.Modeswitches.M5_ResetOSonly := FALSE;
   MOTOR3_No005.PCONF.Modeswitches.sw06 := FALSE;
   MOTOR3_No005.PCONF.Modeswitches.M7_ChgSFviaStop := FALSE;
   MOTOR3_No005.PCONF.Modeswitches.M8_ChgFSviaStop := FALSE;
   MOTOR3_No005.PCONF.Modeswitches.M9_StopIfAutoFail := FALSE;
   MOTOR3_No005.PCONF.Modeswitches.M10_ExtFaultNC := FALSE;
   MOTOR3_No005.PCONF.Modeswitches.sw11 := FALSE;
   MOTOR3_No005.PCONF.Modeswitches.sw12 := FALSE;
   MOTOR3_No005.PCONF.Modeswitches.sw13 := FALSE;
   MOTOR3_No005.PCONF.Modeswitches.sw14 := FALSE;
   MOTOR3_No005.PCONF.Modeswitches.sw15 := FALSE;
   MOTOR3_No005.PCONF.DlyTExtFault := T#0MS;
   MOTOR3_No005.PCONF.DlyTFeedback := T#0MS;
   MOTOR3_No005.PCONF.DlyTActFault := T#0MS;
   MOTOR3_No005.PCONF.DlyTAutoAl := T#0MS;
   MOTOR3_No005.PCONF.DlyTRestart := T#0MS;
   MOTOR3_No005.PCONF.DlyTChgSF := T#0MS;
   MOTOR3_No005.PCONF.DlyTChgFS := T#0MS;
   MOTOR3_No005.PCONF.DlyTChgDirec := T#0MS;
   MOTOR3_No006.System := W#16#0;
   MOTOR3_No006.CmdOS := W#16#0;
   MOTOR3_No006.MirrorCmdOS := W#16#0;
   MOTOR3_No006.Test := W#16#0;
   MOTOR3_No006.AlarmOS := W#16#0;
   MOTOR3_No006.StatusOS := W#16#0;
   MOTOR3_No006.SysStatusOS := W#16#0;
   MOTOR3_No006.Status1 := W#16#0;
   MOTOR3_No006.Status2 := W#16#0;
   MOTOR3_No006.Status3 := B#16#0;
   MOTOR3_No006.InputEdges := B#16#0;
   MOTOR3_No006.AutoEdges := W#16#0;
   MOTOR3_No006.DataTimeExtFault.StartTime := L#0;
   MOTOR3_No006.DataTimeExtFault.StartEdge := FALSE;
   MOTOR3_No006.DataTimeFeedback.StartTime := L#0;
   MOTOR3_No006.DataTimeFeedback.StartEdge := FALSE;
   MOTOR3_No006.DataTimeActFault.StartTime := L#0;
   MOTOR3_No006.DataTimeActFault.StartEdge := FALSE;
   MOTOR3_No006.DataTimeAutoAl.StartTime := L#0;
   MOTOR3_No006.DataTimeAutoAl.StartEdge := FALSE;
   MOTOR3_No006.DataTimeRestart.StartTime := L#0;
   MOTOR3_No006.DataTimeRestart.StartEdge := FALSE;
   MOTOR3_No006.DataTimeChgSF.StartTime := L#0;
   MOTOR3_No006.DataTimeChgSF.StartEdge := FALSE;
   MOTOR3_No006.DataTimeChgFS.StartTime := L#0;
   MOTOR3_No006.DataTimeChgFS.StartEdge := FALSE;
   MOTOR3_No006.DataTimeChgDirec.StartTime := L#0;
   MOTOR3_No006.DataTimeChgDirec.StartEdge := FALSE;
   MOTOR3_No006.PCONF.Modeswitches.M0_ConstantOut := FALSE;
   MOTOR3_No006.PCONF.Modeswitches.M1_AutoManLoc := FALSE;
   MOTOR3_No006.PCONF.Modeswitches.M2_NoActFeedFault := FALSE;
   MOTOR3_No006.PCONF.Modeswitches.M3_NoStopIfFault := FALSE;
   MOTOR3_No006.PCONF.Modeswitches.M4_RestrtAftBlack := FALSE;
   MOTOR3_No006.PCONF.Modeswitches.M5_ResetOSonly := FALSE;
   MOTOR3_No006.PCONF.Modeswitches.sw06 := FALSE;
   MOTOR3_No006.PCONF.Modeswitches.M7_ChgSFviaStop := FALSE;
   MOTOR3_No006.PCONF.Modeswitches.M8_ChgFSviaStop := FALSE;
   MOTOR3_No006.PCONF.Modeswitches.M9_StopIfAutoFail := FALSE;
   MOTOR3_No006.PCONF.Modeswitches.M10_ExtFaultNC := FALSE;
   MOTOR3_No006.PCONF.Modeswitches.sw11 := FALSE;
   MOTOR3_No006.PCONF.Modeswitches.sw12 := FALSE;
   MOTOR3_No006.PCONF.Modeswitches.sw13 := FALSE;
   MOTOR3_No006.PCONF.Modeswitches.sw14 := FALSE;
   MOTOR3_No006.PCONF.Modeswitches.sw15 := FALSE;
   MOTOR3_No006.PCONF.DlyTExtFault := T#0MS;
   MOTOR3_No006.PCONF.DlyTFeedback := T#0MS;
   MOTOR3_No006.PCONF.DlyTActFault := T#0MS;
   MOTOR3_No006.PCONF.DlyTAutoAl := T#0MS;
   MOTOR3_No006.PCONF.DlyTRestart := T#0MS;
   MOTOR3_No006.PCONF.DlyTChgSF := T#0MS;
   MOTOR3_No006.PCONF.DlyTChgFS := T#0MS;
   MOTOR3_No006.PCONF.DlyTChgDirec := T#0MS;
   MOTOR3_No007.System := W#16#0;
   MOTOR3_No007.CmdOS := W#16#0;
   MOTOR3_No007.MirrorCmdOS := W#16#0;
   MOTOR3_No007.Test := W#16#0;
   MOTOR3_No007.AlarmOS := W#16#0;
   MOTOR3_No007.StatusOS := W#16#0;
   MOTOR3_No007.SysStatusOS := W#16#0;
   MOTOR3_No007.Status1 := W#16#0;
   MOTOR3_No007.Status2 := W#16#0;
   MOTOR3_No007.Status3 := B#16#0;
   MOTOR3_No007.InputEdges := B#16#0;
   MOTOR3_No007.AutoEdges := W#16#0;
   MOTOR3_No007.DataTimeExtFault.StartTime := L#0;
   MOTOR3_No007.DataTimeExtFault.StartEdge := FALSE;
   MOTOR3_No007.DataTimeFeedback.StartTime := L#0;
   MOTOR3_No007.DataTimeFeedback.StartEdge := FALSE;
   MOTOR3_No007.DataTimeActFault.StartTime := L#0;
   MOTOR3_No007.DataTimeActFault.StartEdge := FALSE;
   MOTOR3_No007.DataTimeAutoAl.StartTime := L#0;
   MOTOR3_No007.DataTimeAutoAl.StartEdge := FALSE;
   MOTOR3_No007.DataTimeRestart.StartTime := L#0;
   MOTOR3_No007.DataTimeRestart.StartEdge := FALSE;
   MOTOR3_No007.DataTimeChgSF.StartTime := L#0;
   MOTOR3_No007.DataTimeChgSF.StartEdge := FALSE;
   MOTOR3_No007.DataTimeChgFS.StartTime := L#0;
   MOTOR3_No007.DataTimeChgFS.StartEdge := FALSE;
   MOTOR3_No007.DataTimeChgDirec.StartTime := L#0;
   MOTOR3_No007.DataTimeChgDirec.StartEdge := FALSE;
   MOTOR3_No007.PCONF.Modeswitches.M0_ConstantOut := FALSE;
   MOTOR3_No007.PCONF.Modeswitches.M1_AutoManLoc := FALSE;
   MOTOR3_No007.PCONF.Modeswitches.M2_NoActFeedFault := FALSE;
   MOTOR3_No007.PCONF.Modeswitches.M3_NoStopIfFault := FALSE;
   MOTOR3_No007.PCONF.Modeswitches.M4_RestrtAftBlack := FALSE;
   MOTOR3_No007.PCONF.Modeswitches.M5_ResetOSonly := FALSE;
   MOTOR3_No007.PCONF.Modeswitches.sw06 := FALSE;
   MOTOR3_No007.PCONF.Modeswitches.M7_ChgSFviaStop := FALSE;
   MOTOR3_No007.PCONF.Modeswitches.M8_ChgFSviaStop := FALSE;
   MOTOR3_No007.PCONF.Modeswitches.M9_StopIfAutoFail := FALSE;
   MOTOR3_No007.PCONF.Modeswitches.M10_ExtFaultNC := FALSE;
   MOTOR3_No007.PCONF.Modeswitches.sw11 := FALSE;
   MOTOR3_No007.PCONF.Modeswitches.sw12 := FALSE;
   MOTOR3_No007.PCONF.Modeswitches.sw13 := FALSE;
   MOTOR3_No007.PCONF.Modeswitches.sw14 := FALSE;
   MOTOR3_No007.PCONF.Modeswitches.sw15 := FALSE;
   MOTOR3_No007.PCONF.DlyTExtFault := T#0MS;
   MOTOR3_No007.PCONF.DlyTFeedback := T#0MS;
   MOTOR3_No007.PCONF.DlyTActFault := T#0MS;
   MOTOR3_No007.PCONF.DlyTAutoAl := T#0MS;
   MOTOR3_No007.PCONF.DlyTRestart := T#0MS;
   MOTOR3_No007.PCONF.DlyTChgSF := T#0MS;
   MOTOR3_No007.PCONF.DlyTChgFS := T#0MS;
   MOTOR3_No007.PCONF.DlyTChgDirec := T#0MS;
   MOTOR3_No008.System := W#16#0;
   MOTOR3_No008.CmdOS := W#16#0;
   MOTOR3_No008.MirrorCmdOS := W#16#0;
   MOTOR3_No008.Test := W#16#0;
   MOTOR3_No008.AlarmOS := W#16#0;
   MOTOR3_No008.StatusOS := W#16#0;
   MOTOR3_No008.SysStatusOS := W#16#0;
   MOTOR3_No008.Status1 := W#16#0;
   MOTOR3_No008.Status2 := W#16#0;
   MOTOR3_No008.Status3 := B#16#0;
   MOTOR3_No008.InputEdges := B#16#0;
   MOTOR3_No008.AutoEdges := W#16#0;
   MOTOR3_No008.DataTimeExtFault.StartTime := L#0;
   MOTOR3_No008.DataTimeExtFault.StartEdge := FALSE;
   MOTOR3_No008.DataTimeFeedback.StartTime := L#0;
   MOTOR3_No008.DataTimeFeedback.StartEdge := FALSE;
   MOTOR3_No008.DataTimeActFault.StartTime := L#0;
   MOTOR3_No008.DataTimeActFault.StartEdge := FALSE;
   MOTOR3_No008.DataTimeAutoAl.StartTime := L#0;
   MOTOR3_No008.DataTimeAutoAl.StartEdge := FALSE;
   MOTOR3_No008.DataTimeRestart.StartTime := L#0;
   MOTOR3_No008.DataTimeRestart.StartEdge := FALSE;
   MOTOR3_No008.DataTimeChgSF.StartTime := L#0;
   MOTOR3_No008.DataTimeChgSF.StartEdge := FALSE;
   MOTOR3_No008.DataTimeChgFS.StartTime := L#0;
   MOTOR3_No008.DataTimeChgFS.StartEdge := FALSE;
   MOTOR3_No008.DataTimeChgDirec.StartTime := L#0;
   MOTOR3_No008.DataTimeChgDirec.StartEdge := FALSE;
   MOTOR3_No008.PCONF.Modeswitches.M0_ConstantOut := FALSE;
   MOTOR3_No008.PCONF.Modeswitches.M1_AutoManLoc := FALSE;
   MOTOR3_No008.PCONF.Modeswitches.M2_NoActFeedFault := FALSE;
   MOTOR3_No008.PCONF.Modeswitches.M3_NoStopIfFault := FALSE;
   MOTOR3_No008.PCONF.Modeswitches.M4_RestrtAftBlack := FALSE;
   MOTOR3_No008.PCONF.Modeswitches.M5_ResetOSonly := FALSE;
   MOTOR3_No008.PCONF.Modeswitches.sw06 := FALSE;
   MOTOR3_No008.PCONF.Modeswitches.M7_ChgSFviaStop := FALSE;
   MOTOR3_No008.PCONF.Modeswitches.M8_ChgFSviaStop := FALSE;
   MOTOR3_No008.PCONF.Modeswitches.M9_StopIfAutoFail := FALSE;
   MOTOR3_No008.PCONF.Modeswitches.M10_ExtFaultNC := FALSE;
   MOTOR3_No008.PCONF.Modeswitches.sw11 := FALSE;
   MOTOR3_No008.PCONF.Modeswitches.sw12 := FALSE;
   MOTOR3_No008.PCONF.Modeswitches.sw13 := FALSE;
   MOTOR3_No008.PCONF.Modeswitches.sw14 := FALSE;
   MOTOR3_No008.PCONF.Modeswitches.sw15 := FALSE;
   MOTOR3_No008.PCONF.DlyTExtFault := T#0MS;
   MOTOR3_No008.PCONF.DlyTFeedback := T#0MS;
   MOTOR3_No008.PCONF.DlyTActFault := T#0MS;
   MOTOR3_No008.PCONF.DlyTAutoAl := T#0MS;
   MOTOR3_No008.PCONF.DlyTRestart := T#0MS;
   MOTOR3_No008.PCONF.DlyTChgSF := T#0MS;
   MOTOR3_No008.PCONF.DlyTChgFS := T#0MS;
   MOTOR3_No008.PCONF.DlyTChgDirec := T#0MS;
   MOTOR3_No009.System := W#16#0;
   MOTOR3_No009.CmdOS := W#16#0;
   MOTOR3_No009.MirrorCmdOS := W#16#0;
   MOTOR3_No009.Test := W#16#0;
   MOTOR3_No009.AlarmOS := W#16#0;
   MOTOR3_No009.StatusOS := W#16#0;
   MOTOR3_No009.SysStatusOS := W#16#0;
   MOTOR3_No009.Status1 := W#16#0;
   MOTOR3_No009.Status2 := W#16#0;
   MOTOR3_No009.Status3 := B#16#0;
   MOTOR3_No009.InputEdges := B#16#0;
   MOTOR3_No009.AutoEdges := W#16#0;
   MOTOR3_No009.DataTimeExtFault.StartTime := L#0;
   MOTOR3_No009.DataTimeExtFault.StartEdge := FALSE;
   MOTOR3_No009.DataTimeFeedback.StartTime := L#0;
   MOTOR3_No009.DataTimeFeedback.StartEdge := FALSE;
   MOTOR3_No009.DataTimeActFault.StartTime := L#0;
   MOTOR3_No009.DataTimeActFault.StartEdge := FALSE;
   MOTOR3_No009.DataTimeAutoAl.StartTime := L#0;
   MOTOR3_No009.DataTimeAutoAl.StartEdge := FALSE;
   MOTOR3_No009.DataTimeRestart.StartTime := L#0;
   MOTOR3_No009.DataTimeRestart.StartEdge := FALSE;
   MOTOR3_No009.DataTimeChgSF.StartTime := L#0;
   MOTOR3_No009.DataTimeChgSF.StartEdge := FALSE;
   MOTOR3_No009.DataTimeChgFS.StartTime := L#0;
   MOTOR3_No009.DataTimeChgFS.StartEdge := FALSE;
   MOTOR3_No009.DataTimeChgDirec.StartTime := L#0;
   MOTOR3_No009.DataTimeChgDirec.StartEdge := FALSE;
   MOTOR3_No009.PCONF.Modeswitches.M0_ConstantOut := FALSE;
   MOTOR3_No009.PCONF.Modeswitches.M1_AutoManLoc := FALSE;
   MOTOR3_No009.PCONF.Modeswitches.M2_NoActFeedFault := FALSE;
   MOTOR3_No009.PCONF.Modeswitches.M3_NoStopIfFault := FALSE;
   MOTOR3_No009.PCONF.Modeswitches.M4_RestrtAftBlack := FALSE;
   MOTOR3_No009.PCONF.Modeswitches.M5_ResetOSonly := FALSE;
   MOTOR3_No009.PCONF.Modeswitches.sw06 := FALSE;
   MOTOR3_No009.PCONF.Modeswitches.M7_ChgSFviaStop := FALSE;
   MOTOR3_No009.PCONF.Modeswitches.M8_ChgFSviaStop := FALSE;
   MOTOR3_No009.PCONF.Modeswitches.M9_StopIfAutoFail := FALSE;
   MOTOR3_No009.PCONF.Modeswitches.M10_ExtFaultNC := FALSE;
   MOTOR3_No009.PCONF.Modeswitches.sw11 := FALSE;
   MOTOR3_No009.PCONF.Modeswitches.sw12 := FALSE;
   MOTOR3_No009.PCONF.Modeswitches.sw13 := FALSE;
   MOTOR3_No009.PCONF.Modeswitches.sw14 := FALSE;
   MOTOR3_No009.PCONF.Modeswitches.sw15 := FALSE;
   MOTOR3_No009.PCONF.DlyTExtFault := T#0MS;
   MOTOR3_No009.PCONF.DlyTFeedback := T#0MS;
   MOTOR3_No009.PCONF.DlyTActFault := T#0MS;
   MOTOR3_No009.PCONF.DlyTAutoAl := T#0MS;
   MOTOR3_No009.PCONF.DlyTRestart := T#0MS;
   MOTOR3_No009.PCONF.DlyTChgSF := T#0MS;
   MOTOR3_No009.PCONF.DlyTChgFS := T#0MS;
   MOTOR3_No009.PCONF.DlyTChgDirec := T#0MS;
   MOTOR3_No010.System := W#16#0;
   MOTOR3_No010.CmdOS := W#16#0;
   MOTOR3_No010.MirrorCmdOS := W#16#0;
   MOTOR3_No010.Test := W#16#0;
   MOTOR3_No010.AlarmOS := W#16#0;
   MOTOR3_No010.StatusOS := W#16#0;
   MOTOR3_No010.SysStatusOS := W#16#0;
   MOTOR3_No010.Status1 := W#16#0;
   MOTOR3_No010.Status2 := W#16#0;
   MOTOR3_No010.Status3 := B#16#0;
   MOTOR3_No010.InputEdges := B#16#0;
   MOTOR3_No010.AutoEdges := W#16#0;
   MOTOR3_No010.DataTimeExtFault.StartTime := L#0;
   MOTOR3_No010.DataTimeExtFault.StartEdge := FALSE;
   MOTOR3_No010.DataTimeFeedback.StartTime := L#0;
   MOTOR3_No010.DataTimeFeedback.StartEdge := FALSE;
   MOTOR3_No010.DataTimeActFault.StartTime := L#0;
   MOTOR3_No010.DataTimeActFault.StartEdge := FALSE;
   MOTOR3_No010.DataTimeAutoAl.StartTime := L#0;
   MOTOR3_No010.DataTimeAutoAl.StartEdge := FALSE;
   MOTOR3_No010.DataTimeRestart.StartTime := L#0;
   MOTOR3_No010.DataTimeRestart.StartEdge := FALSE;
   MOTOR3_No010.DataTimeChgSF.StartTime := L#0;
   MOTOR3_No010.DataTimeChgSF.StartEdge := FALSE;
   MOTOR3_No010.DataTimeChgFS.StartTime := L#0;
   MOTOR3_No010.DataTimeChgFS.StartEdge := FALSE;
   MOTOR3_No010.DataTimeChgDirec.StartTime := L#0;
   MOTOR3_No010.DataTimeChgDirec.StartEdge := FALSE;
   MOTOR3_No010.PCONF.Modeswitches.M0_ConstantOut := FALSE;
   MOTOR3_No010.PCONF.Modeswitches.M1_AutoManLoc := FALSE;
   MOTOR3_No010.PCONF.Modeswitches.M2_NoActFeedFault := FALSE;
   MOTOR3_No010.PCONF.Modeswitches.M3_NoStopIfFault := FALSE;
   MOTOR3_No010.PCONF.Modeswitches.M4_RestrtAftBlack := FALSE;
   MOTOR3_No010.PCONF.Modeswitches.M5_ResetOSonly := FALSE;
   MOTOR3_No010.PCONF.Modeswitches.sw06 := FALSE;
   MOTOR3_No010.PCONF.Modeswitches.M7_ChgSFviaStop := FALSE;
   MOTOR3_No010.PCONF.Modeswitches.M8_ChgFSviaStop := FALSE;
   MOTOR3_No010.PCONF.Modeswitches.M9_StopIfAutoFail := FALSE;
   MOTOR3_No010.PCONF.Modeswitches.M10_ExtFaultNC := FALSE;
   MOTOR3_No010.PCONF.Modeswitches.sw11 := FALSE;
   MOTOR3_No010.PCONF.Modeswitches.sw12 := FALSE;
   MOTOR3_No010.PCONF.Modeswitches.sw13 := FALSE;
   MOTOR3_No010.PCONF.Modeswitches.sw14 := FALSE;
   MOTOR3_No010.PCONF.Modeswitches.sw15 := FALSE;
   MOTOR3_No010.PCONF.DlyTExtFault := T#0MS;
   MOTOR3_No010.PCONF.DlyTFeedback := T#0MS;
   MOTOR3_No010.PCONF.DlyTActFault := T#0MS;
   MOTOR3_No010.PCONF.DlyTAutoAl := T#0MS;
   MOTOR3_No010.PCONF.DlyTRestart := T#0MS;
   MOTOR3_No010.PCONF.DlyTChgSF := T#0MS;
   MOTOR3_No010.PCONF.DlyTChgFS := T#0MS;
   MOTOR3_No010.PCONF.DlyTChgDirec := T#0MS;
   MOTOR3_No011.System := W#16#0;
   MOTOR3_No011.CmdOS := W#16#0;
   MOTOR3_No011.MirrorCmdOS := W#16#0;
   MOTOR3_No011.Test := W#16#0;
   MOTOR3_No011.AlarmOS := W#16#0;
   MOTOR3_No011.StatusOS := W#16#0;
   MOTOR3_No011.SysStatusOS := W#16#0;
   MOTOR3_No011.Status1 := W#16#0;
   MOTOR3_No011.Status2 := W#16#0;
   MOTOR3_No011.Status3 := B#16#0;
   MOTOR3_No011.InputEdges := B#16#0;
   MOTOR3_No011.AutoEdges := W#16#0;
   MOTOR3_No011.DataTimeExtFault.StartTime := L#0;
   MOTOR3_No011.DataTimeExtFault.StartEdge := FALSE;
   MOTOR3_No011.DataTimeFeedback.StartTime := L#0;
   MOTOR3_No011.DataTimeFeedback.StartEdge := FALSE;
   MOTOR3_No011.DataTimeActFault.StartTime := L#0;
   MOTOR3_No011.DataTimeActFault.StartEdge := FALSE;
   MOTOR3_No011.DataTimeAutoAl.StartTime := L#0;
   MOTOR3_No011.DataTimeAutoAl.StartEdge := FALSE;
   MOTOR3_No011.DataTimeRestart.StartTime := L#0;
   MOTOR3_No011.DataTimeRestart.StartEdge := FALSE;
   MOTOR3_No011.DataTimeChgSF.StartTime := L#0;
   MOTOR3_No011.DataTimeChgSF.StartEdge := FALSE;
   MOTOR3_No011.DataTimeChgFS.StartTime := L#0;
   MOTOR3_No011.DataTimeChgFS.StartEdge := FALSE;
   MOTOR3_No011.DataTimeChgDirec.StartTime := L#0;
   MOTOR3_No011.DataTimeChgDirec.StartEdge := FALSE;
   MOTOR3_No011.PCONF.Modeswitches.M0_ConstantOut := FALSE;
   MOTOR3_No011.PCONF.Modeswitches.M1_AutoManLoc := FALSE;
   MOTOR3_No011.PCONF.Modeswitches.M2_NoActFeedFault := FALSE;
   MOTOR3_No011.PCONF.Modeswitches.M3_NoStopIfFault := FALSE;
   MOTOR3_No011.PCONF.Modeswitches.M4_RestrtAftBlack := FALSE;
   MOTOR3_No011.PCONF.Modeswitches.M5_ResetOSonly := FALSE;
   MOTOR3_No011.PCONF.Modeswitches.sw06 := FALSE;
   MOTOR3_No011.PCONF.Modeswitches.M7_ChgSFviaStop := FALSE;
   MOTOR3_No011.PCONF.Modeswitches.M8_ChgFSviaStop := FALSE;
   MOTOR3_No011.PCONF.Modeswitches.M9_StopIfAutoFail := FALSE;
   MOTOR3_No011.PCONF.Modeswitches.M10_ExtFaultNC := FALSE;
   MOTOR3_No011.PCONF.Modeswitches.sw11 := FALSE;
   MOTOR3_No011.PCONF.Modeswitches.sw12 := FALSE;
   MOTOR3_No011.PCONF.Modeswitches.sw13 := FALSE;
   MOTOR3_No011.PCONF.Modeswitches.sw14 := FALSE;
   MOTOR3_No011.PCONF.Modeswitches.sw15 := FALSE;
   MOTOR3_No011.PCONF.DlyTExtFault := T#0MS;
   MOTOR3_No011.PCONF.DlyTFeedback := T#0MS;
   MOTOR3_No011.PCONF.DlyTActFault := T#0MS;
   MOTOR3_No011.PCONF.DlyTAutoAl := T#0MS;
   MOTOR3_No011.PCONF.DlyTRestart := T#0MS;
   MOTOR3_No011.PCONF.DlyTChgSF := T#0MS;
   MOTOR3_No011.PCONF.DlyTChgFS := T#0MS;
   MOTOR3_No011.PCONF.DlyTChgDirec := T#0MS;
   MOTOR3_No012.System := W#16#0;
   MOTOR3_No012.CmdOS := W#16#0;
   MOTOR3_No012.MirrorCmdOS := W#16#0;
   MOTOR3_No012.Test := W#16#0;
   MOTOR3_No012.AlarmOS := W#16#0;
   MOTOR3_No012.StatusOS := W#16#0;
   MOTOR3_No012.SysStatusOS := W#16#0;
   MOTOR3_No012.Status1 := W#16#0;
   MOTOR3_No012.Status2 := W#16#0;
   MOTOR3_No012.Status3 := B#16#0;
   MOTOR3_No012.InputEdges := B#16#0;
   MOTOR3_No012.AutoEdges := W#16#0;
   MOTOR3_No012.DataTimeExtFault.StartTime := L#0;
   MOTOR3_No012.DataTimeExtFault.StartEdge := FALSE;
   MOTOR3_No012.DataTimeFeedback.StartTime := L#0;
   MOTOR3_No012.DataTimeFeedback.StartEdge := FALSE;
   MOTOR3_No012.DataTimeActFault.StartTime := L#0;
   MOTOR3_No012.DataTimeActFault.StartEdge := FALSE;
   MOTOR3_No012.DataTimeAutoAl.StartTime := L#0;
   MOTOR3_No012.DataTimeAutoAl.StartEdge := FALSE;
   MOTOR3_No012.DataTimeRestart.StartTime := L#0;
   MOTOR3_No012.DataTimeRestart.StartEdge := FALSE;
   MOTOR3_No012.DataTimeChgSF.StartTime := L#0;
   MOTOR3_No012.DataTimeChgSF.StartEdge := FALSE;
   MOTOR3_No012.DataTimeChgFS.StartTime := L#0;
   MOTOR3_No012.DataTimeChgFS.StartEdge := FALSE;
   MOTOR3_No012.DataTimeChgDirec.StartTime := L#0;
   MOTOR3_No012.DataTimeChgDirec.StartEdge := FALSE;
   MOTOR3_No012.PCONF.Modeswitches.M0_ConstantOut := FALSE;
   MOTOR3_No012.PCONF.Modeswitches.M1_AutoManLoc := FALSE;
   MOTOR3_No012.PCONF.Modeswitches.M2_NoActFeedFault := FALSE;
   MOTOR3_No012.PCONF.Modeswitches.M3_NoStopIfFault := FALSE;
   MOTOR3_No012.PCONF.Modeswitches.M4_RestrtAftBlack := FALSE;
   MOTOR3_No012.PCONF.Modeswitches.M5_ResetOSonly := FALSE;
   MOTOR3_No012.PCONF.Modeswitches.sw06 := FALSE;
   MOTOR3_No012.PCONF.Modeswitches.M7_ChgSFviaStop := FALSE;
   MOTOR3_No012.PCONF.Modeswitches.M8_ChgFSviaStop := FALSE;
   MOTOR3_No012.PCONF.Modeswitches.M9_StopIfAutoFail := FALSE;
   MOTOR3_No012.PCONF.Modeswitches.M10_ExtFaultNC := FALSE;
   MOTOR3_No012.PCONF.Modeswitches.sw11 := FALSE;
   MOTOR3_No012.PCONF.Modeswitches.sw12 := FALSE;
   MOTOR3_No012.PCONF.Modeswitches.sw13 := FALSE;
   MOTOR3_No012.PCONF.Modeswitches.sw14 := FALSE;
   MOTOR3_No012.PCONF.Modeswitches.sw15 := FALSE;
   MOTOR3_No012.PCONF.DlyTExtFault := T#0MS;
   MOTOR3_No012.PCONF.DlyTFeedback := T#0MS;
   MOTOR3_No012.PCONF.DlyTActFault := T#0MS;
   MOTOR3_No012.PCONF.DlyTAutoAl := T#0MS;
   MOTOR3_No012.PCONF.DlyTRestart := T#0MS;
   MOTOR3_No012.PCONF.DlyTChgSF := T#0MS;
   MOTOR3_No012.PCONF.DlyTChgFS := T#0MS;
   MOTOR3_No012.PCONF.DlyTChgDirec := T#0MS;
   MOTOR3_No013.System := W#16#0;
   MOTOR3_No013.CmdOS := W#16#0;
   MOTOR3_No013.MirrorCmdOS := W#16#0;
   MOTOR3_No013.Test := W#16#0;
   MOTOR3_No013.AlarmOS := W#16#0;
   MOTOR3_No013.StatusOS := W#16#0;
   MOTOR3_No013.SysStatusOS := W#16#0;
   MOTOR3_No013.Status1 := W#16#0;
   MOTOR3_No013.Status2 := W#16#0;
   MOTOR3_No013.Status3 := B#16#0;
   MOTOR3_No013.InputEdges := B#16#0;
   MOTOR3_No013.AutoEdges := W#16#0;
   MOTOR3_No013.DataTimeExtFault.StartTime := L#0;
   MOTOR3_No013.DataTimeExtFault.StartEdge := FALSE;
   MOTOR3_No013.DataTimeFeedback.StartTime := L#0;
   MOTOR3_No013.DataTimeFeedback.StartEdge := FALSE;
   MOTOR3_No013.DataTimeActFault.StartTime := L#0;
   MOTOR3_No013.DataTimeActFault.StartEdge := FALSE;
   MOTOR3_No013.DataTimeAutoAl.StartTime := L#0;
   MOTOR3_No013.DataTimeAutoAl.StartEdge := FALSE;
   MOTOR3_No013.DataTimeRestart.StartTime := L#0;
   MOTOR3_No013.DataTimeRestart.StartEdge := FALSE;
   MOTOR3_No013.DataTimeChgSF.StartTime := L#0;
   MOTOR3_No013.DataTimeChgSF.StartEdge := FALSE;
   MOTOR3_No013.DataTimeChgFS.StartTime := L#0;
   MOTOR3_No013.DataTimeChgFS.StartEdge := FALSE;
   MOTOR3_No013.DataTimeChgDirec.StartTime := L#0;
   MOTOR3_No013.DataTimeChgDirec.StartEdge := FALSE;
   MOTOR3_No013.PCONF.Modeswitches.M0_ConstantOut := FALSE;
   MOTOR3_No013.PCONF.Modeswitches.M1_AutoManLoc := FALSE;
   MOTOR3_No013.PCONF.Modeswitches.M2_NoActFeedFault := FALSE;
   MOTOR3_No013.PCONF.Modeswitches.M3_NoStopIfFault := FALSE;
   MOTOR3_No013.PCONF.Modeswitches.M4_RestrtAftBlack := FALSE;
   MOTOR3_No013.PCONF.Modeswitches.M5_ResetOSonly := FALSE;
   MOTOR3_No013.PCONF.Modeswitches.sw06 := FALSE;
   MOTOR3_No013.PCONF.Modeswitches.M7_ChgSFviaStop := FALSE;
   MOTOR3_No013.PCONF.Modeswitches.M8_ChgFSviaStop := FALSE;
   MOTOR3_No013.PCONF.Modeswitches.M9_StopIfAutoFail := FALSE;
   MOTOR3_No013.PCONF.Modeswitches.M10_ExtFaultNC := FALSE;
   MOTOR3_No013.PCONF.Modeswitches.sw11 := FALSE;
   MOTOR3_No013.PCONF.Modeswitches.sw12 := FALSE;
   MOTOR3_No013.PCONF.Modeswitches.sw13 := FALSE;
   MOTOR3_No013.PCONF.Modeswitches.sw14 := FALSE;
   MOTOR3_No013.PCONF.Modeswitches.sw15 := FALSE;
   MOTOR3_No013.PCONF.DlyTExtFault := T#0MS;
   MOTOR3_No013.PCONF.DlyTFeedback := T#0MS;
   MOTOR3_No013.PCONF.DlyTActFault := T#0MS;
   MOTOR3_No013.PCONF.DlyTAutoAl := T#0MS;
   MOTOR3_No013.PCONF.DlyTRestart := T#0MS;
   MOTOR3_No013.PCONF.DlyTChgSF := T#0MS;
   MOTOR3_No013.PCONF.DlyTChgFS := T#0MS;
   MOTOR3_No013.PCONF.DlyTChgDirec := T#0MS;
   MOTOR3_No014.System := W#16#0;
   MOTOR3_No014.CmdOS := W#16#0;
   MOTOR3_No014.MirrorCmdOS := W#16#0;
   MOTOR3_No014.Test := W#16#0;
   MOTOR3_No014.AlarmOS := W#16#0;
   MOTOR3_No014.StatusOS := W#16#0;
   MOTOR3_No014.SysStatusOS := W#16#0;
   MOTOR3_No014.Status1 := W#16#0;
   MOTOR3_No014.Status2 := W#16#0;
   MOTOR3_No014.Status3 := B#16#0;
   MOTOR3_No014.InputEdges := B#16#0;
   MOTOR3_No014.AutoEdges := W#16#0;
   MOTOR3_No014.DataTimeExtFault.StartTime := L#0;
   MOTOR3_No014.DataTimeExtFault.StartEdge := FALSE;
   MOTOR3_No014.DataTimeFeedback.StartTime := L#0;
   MOTOR3_No014.DataTimeFeedback.StartEdge := FALSE;
   MOTOR3_No014.DataTimeActFault.StartTime := L#0;
   MOTOR3_No014.DataTimeActFault.StartEdge := FALSE;
   MOTOR3_No014.DataTimeAutoAl.StartTime := L#0;
   MOTOR3_No014.DataTimeAutoAl.StartEdge := FALSE;
   MOTOR3_No014.DataTimeRestart.StartTime := L#0;
   MOTOR3_No014.DataTimeRestart.StartEdge := FALSE;
   MOTOR3_No014.DataTimeChgSF.StartTime := L#0;
   MOTOR3_No014.DataTimeChgSF.StartEdge := FALSE;
   MOTOR3_No014.DataTimeChgFS.StartTime := L#0;
   MOTOR3_No014.DataTimeChgFS.StartEdge := FALSE;
   MOTOR3_No014.DataTimeChgDirec.StartTime := L#0;
   MOTOR3_No014.DataTimeChgDirec.StartEdge := FALSE;
   MOTOR3_No014.PCONF.Modeswitches.M0_ConstantOut := FALSE;
   MOTOR3_No014.PCONF.Modeswitches.M1_AutoManLoc := FALSE;
   MOTOR3_No014.PCONF.Modeswitches.M2_NoActFeedFault := FALSE;
   MOTOR3_No014.PCONF.Modeswitches.M3_NoStopIfFault := FALSE;
   MOTOR3_No014.PCONF.Modeswitches.M4_RestrtAftBlack := FALSE;
   MOTOR3_No014.PCONF.Modeswitches.M5_ResetOSonly := FALSE;
   MOTOR3_No014.PCONF.Modeswitches.sw06 := FALSE;
   MOTOR3_No014.PCONF.Modeswitches.M7_ChgSFviaStop := FALSE;
   MOTOR3_No014.PCONF.Modeswitches.M8_ChgFSviaStop := FALSE;
   MOTOR3_No014.PCONF.Modeswitches.M9_StopIfAutoFail := FALSE;
   MOTOR3_No014.PCONF.Modeswitches.M10_ExtFaultNC := FALSE;
   MOTOR3_No014.PCONF.Modeswitches.sw11 := FALSE;
   MOTOR3_No014.PCONF.Modeswitches.sw12 := FALSE;
   MOTOR3_No014.PCONF.Modeswitches.sw13 := FALSE;
   MOTOR3_No014.PCONF.Modeswitches.sw14 := FALSE;
   MOTOR3_No014.PCONF.Modeswitches.sw15 := FALSE;
   MOTOR3_No014.PCONF.DlyTExtFault := T#0MS;
   MOTOR3_No014.PCONF.DlyTFeedback := T#0MS;
   MOTOR3_No014.PCONF.DlyTActFault := T#0MS;
   MOTOR3_No014.PCONF.DlyTAutoAl := T#0MS;
   MOTOR3_No014.PCONF.DlyTRestart := T#0MS;
   MOTOR3_No014.PCONF.DlyTChgSF := T#0MS;
   MOTOR3_No014.PCONF.DlyTChgFS := T#0MS;
   MOTOR3_No014.PCONF.DlyTChgDirec := T#0MS;
   MOTOR3_No015.System := W#16#0;
   MOTOR3_No015.CmdOS := W#16#0;
   MOTOR3_No015.MirrorCmdOS := W#16#0;
   MOTOR3_No015.Test := W#16#0;
   MOTOR3_No015.AlarmOS := W#16#0;
   MOTOR3_No015.StatusOS := W#16#0;
   MOTOR3_No015.SysStatusOS := W#16#0;
   MOTOR3_No015.Status1 := W#16#0;
   MOTOR3_No015.Status2 := W#16#0;
   MOTOR3_No015.Status3 := B#16#0;
   MOTOR3_No015.InputEdges := B#16#0;
   MOTOR3_No015.AutoEdges := W#16#0;
   MOTOR3_No015.DataTimeExtFault.StartTime := L#0;
   MOTOR3_No015.DataTimeExtFault.StartEdge := FALSE;
   MOTOR3_No015.DataTimeFeedback.StartTime := L#0;
   MOTOR3_No015.DataTimeFeedback.StartEdge := FALSE;
   MOTOR3_No015.DataTimeActFault.StartTime := L#0;
   MOTOR3_No015.DataTimeActFault.StartEdge := FALSE;
   MOTOR3_No015.DataTimeAutoAl.StartTime := L#0;
   MOTOR3_No015.DataTimeAutoAl.StartEdge := FALSE;
   MOTOR3_No015.DataTimeRestart.StartTime := L#0;
   MOTOR3_No015.DataTimeRestart.StartEdge := FALSE;
   MOTOR3_No015.DataTimeChgSF.StartTime := L#0;
   MOTOR3_No015.DataTimeChgSF.StartEdge := FALSE;
   MOTOR3_No015.DataTimeChgFS.StartTime := L#0;
   MOTOR3_No015.DataTimeChgFS.StartEdge := FALSE;
   MOTOR3_No015.DataTimeChgDirec.StartTime := L#0;
   MOTOR3_No015.DataTimeChgDirec.StartEdge := FALSE;
   MOTOR3_No015.PCONF.Modeswitches.M0_ConstantOut := FALSE;
   MOTOR3_No015.PCONF.Modeswitches.M1_AutoManLoc := FALSE;
   MOTOR3_No015.PCONF.Modeswitches.M2_NoActFeedFault := FALSE;
   MOTOR3_No015.PCONF.Modeswitches.M3_NoStopIfFault := FALSE;
   MOTOR3_No015.PCONF.Modeswitches.M4_RestrtAftBlack := FALSE;
   MOTOR3_No015.PCONF.Modeswitches.M5_ResetOSonly := FALSE;
   MOTOR3_No015.PCONF.Modeswitches.sw06 := FALSE;
   MOTOR3_No015.PCONF.Modeswitches.M7_ChgSFviaStop := FALSE;
   MOTOR3_No015.PCONF.Modeswitches.M8_ChgFSviaStop := FALSE;
   MOTOR3_No015.PCONF.Modeswitches.M9_StopIfAutoFail := FALSE;
   MOTOR3_No015.PCONF.Modeswitches.M10_ExtFaultNC := FALSE;
   MOTOR3_No015.PCONF.Modeswitches.sw11 := FALSE;
   MOTOR3_No015.PCONF.Modeswitches.sw12 := FALSE;
   MOTOR3_No015.PCONF.Modeswitches.sw13 := FALSE;
   MOTOR3_No015.PCONF.Modeswitches.sw14 := FALSE;
   MOTOR3_No015.PCONF.Modeswitches.sw15 := FALSE;
   MOTOR3_No015.PCONF.DlyTExtFault := T#0MS;
   MOTOR3_No015.PCONF.DlyTFeedback := T#0MS;
   MOTOR3_No015.PCONF.DlyTActFault := T#0MS;
   MOTOR3_No015.PCONF.DlyTAutoAl := T#0MS;
   MOTOR3_No015.PCONF.DlyTRestart := T#0MS;
   MOTOR3_No015.PCONF.DlyTChgSF := T#0MS;
   MOTOR3_No015.PCONF.DlyTChgFS := T#0MS;
   MOTOR3_No015.PCONF.DlyTChgDirec := T#0MS;
   MOTOR3_No016.System := W#16#0;
   MOTOR3_No016.CmdOS := W#16#0;
   MOTOR3_No016.MirrorCmdOS := W#16#0;
   MOTOR3_No016.Test := W#16#0;
   MOTOR3_No016.AlarmOS := W#16#0;
   MOTOR3_No016.StatusOS := W#16#0;
   MOTOR3_No016.SysStatusOS := W#16#0;
   MOTOR3_No016.Status1 := W#16#0;
   MOTOR3_No016.Status2 := W#16#0;
   MOTOR3_No016.Status3 := B#16#0;
   MOTOR3_No016.InputEdges := B#16#0;
   MOTOR3_No016.AutoEdges := W#16#0;
   MOTOR3_No016.DataTimeExtFault.StartTime := L#0;
   MOTOR3_No016.DataTimeExtFault.StartEdge := FALSE;
   MOTOR3_No016.DataTimeFeedback.StartTime := L#0;
   MOTOR3_No016.DataTimeFeedback.StartEdge := FALSE;
   MOTOR3_No016.DataTimeActFault.StartTime := L#0;
   MOTOR3_No016.DataTimeActFault.StartEdge := FALSE;
   MOTOR3_No016.DataTimeAutoAl.StartTime := L#0;
   MOTOR3_No016.DataTimeAutoAl.StartEdge := FALSE;
   MOTOR3_No016.DataTimeRestart.StartTime := L#0;
   MOTOR3_No016.DataTimeRestart.StartEdge := FALSE;
   MOTOR3_No016.DataTimeChgSF.StartTime := L#0;
   MOTOR3_No016.DataTimeChgSF.StartEdge := FALSE;
   MOTOR3_No016.DataTimeChgFS.StartTime := L#0;
   MOTOR3_No016.DataTimeChgFS.StartEdge := FALSE;
   MOTOR3_No016.DataTimeChgDirec.StartTime := L#0;
   MOTOR3_No016.DataTimeChgDirec.StartEdge := FALSE;
   MOTOR3_No016.PCONF.Modeswitches.M0_ConstantOut := FALSE;
   MOTOR3_No016.PCONF.Modeswitches.M1_AutoManLoc := FALSE;
   MOTOR3_No016.PCONF.Modeswitches.M2_NoActFeedFault := FALSE;
   MOTOR3_No016.PCONF.Modeswitches.M3_NoStopIfFault := FALSE;
   MOTOR3_No016.PCONF.Modeswitches.M4_RestrtAftBlack := FALSE;
   MOTOR3_No016.PCONF.Modeswitches.M5_ResetOSonly := FALSE;
   MOTOR3_No016.PCONF.Modeswitches.sw06 := FALSE;
   MOTOR3_No016.PCONF.Modeswitches.M7_ChgSFviaStop := FALSE;
   MOTOR3_No016.PCONF.Modeswitches.M8_ChgFSviaStop := FALSE;
   MOTOR3_No016.PCONF.Modeswitches.M9_StopIfAutoFail := FALSE;
   MOTOR3_No016.PCONF.Modeswitches.M10_ExtFaultNC := FALSE;
   MOTOR3_No016.PCONF.Modeswitches.sw11 := FALSE;
   MOTOR3_No016.PCONF.Modeswitches.sw12 := FALSE;
   MOTOR3_No016.PCONF.Modeswitches.sw13 := FALSE;
   MOTOR3_No016.PCONF.Modeswitches.sw14 := FALSE;
   MOTOR3_No016.PCONF.Modeswitches.sw15 := FALSE;
   MOTOR3_No016.PCONF.DlyTExtFault := T#0MS;
   MOTOR3_No016.PCONF.DlyTFeedback := T#0MS;
   MOTOR3_No016.PCONF.DlyTActFault := T#0MS;
   MOTOR3_No016.PCONF.DlyTAutoAl := T#0MS;
   MOTOR3_No016.PCONF.DlyTRestart := T#0MS;
   MOTOR3_No016.PCONF.DlyTChgSF := T#0MS;
   MOTOR3_No016.PCONF.DlyTChgFS := T#0MS;
   MOTOR3_No016.PCONF.DlyTChgDirec := T#0MS;
   MOTOR3_No017.System := W#16#0;
   MOTOR3_No017.CmdOS := W#16#0;
   MOTOR3_No017.MirrorCmdOS := W#16#0;
   MOTOR3_No017.Test := W#16#0;
   MOTOR3_No017.AlarmOS := W#16#0;
   MOTOR3_No017.StatusOS := W#16#0;
   MOTOR3_No017.SysStatusOS := W#16#0;
   MOTOR3_No017.Status1 := W#16#0;
   MOTOR3_No017.Status2 := W#16#0;
   MOTOR3_No017.Status3 := B#16#0;
   MOTOR3_No017.InputEdges := B#16#0;
   MOTOR3_No017.AutoEdges := W#16#0;
   MOTOR3_No017.DataTimeExtFault.StartTime := L#0;
   MOTOR3_No017.DataTimeExtFault.StartEdge := FALSE;
   MOTOR3_No017.DataTimeFeedback.StartTime := L#0;
   MOTOR3_No017.DataTimeFeedback.StartEdge := FALSE;
   MOTOR3_No017.DataTimeActFault.StartTime := L#0;
   MOTOR3_No017.DataTimeActFault.StartEdge := FALSE;
   MOTOR3_No017.DataTimeAutoAl.StartTime := L#0;
   MOTOR3_No017.DataTimeAutoAl.StartEdge := FALSE;
   MOTOR3_No017.DataTimeRestart.StartTime := L#0;
   MOTOR3_No017.DataTimeRestart.StartEdge := FALSE;
   MOTOR3_No017.DataTimeChgSF.StartTime := L#0;
   MOTOR3_No017.DataTimeChgSF.StartEdge := FALSE;
   MOTOR3_No017.DataTimeChgFS.StartTime := L#0;
   MOTOR3_No017.DataTimeChgFS.StartEdge := FALSE;
   MOTOR3_No017.DataTimeChgDirec.StartTime := L#0;
   MOTOR3_No017.DataTimeChgDirec.StartEdge := FALSE;
   MOTOR3_No017.PCONF.Modeswitches.M0_ConstantOut := FALSE;
   MOTOR3_No017.PCONF.Modeswitches.M1_AutoManLoc := FALSE;
   MOTOR3_No017.PCONF.Modeswitches.M2_NoActFeedFault := FALSE;
   MOTOR3_No017.PCONF.Modeswitches.M3_NoStopIfFault := FALSE;
   MOTOR3_No017.PCONF.Modeswitches.M4_RestrtAftBlack := FALSE;
   MOTOR3_No017.PCONF.Modeswitches.M5_ResetOSonly := FALSE;
   MOTOR3_No017.PCONF.Modeswitches.sw06 := FALSE;
   MOTOR3_No017.PCONF.Modeswitches.M7_ChgSFviaStop := FALSE;
   MOTOR3_No017.PCONF.Modeswitches.M8_ChgFSviaStop := FALSE;
   MOTOR3_No017.PCONF.Modeswitches.M9_StopIfAutoFail := FALSE;
   MOTOR3_No017.PCONF.Modeswitches.M10_ExtFaultNC := FALSE;
   MOTOR3_No017.PCONF.Modeswitches.sw11 := FALSE;
   MOTOR3_No017.PCONF.Modeswitches.sw12 := FALSE;
   MOTOR3_No017.PCONF.Modeswitches.sw13 := FALSE;
   MOTOR3_No017.PCONF.Modeswitches.sw14 := FALSE;
   MOTOR3_No017.PCONF.Modeswitches.sw15 := FALSE;
   MOTOR3_No017.PCONF.DlyTExtFault := T#0MS;
   MOTOR3_No017.PCONF.DlyTFeedback := T#0MS;
   MOTOR3_No017.PCONF.DlyTActFault := T#0MS;
   MOTOR3_No017.PCONF.DlyTAutoAl := T#0MS;
   MOTOR3_No017.PCONF.DlyTRestart := T#0MS;
   MOTOR3_No017.PCONF.DlyTChgSF := T#0MS;
   MOTOR3_No017.PCONF.DlyTChgFS := T#0MS;
   MOTOR3_No017.PCONF.DlyTChgDirec := T#0MS;
   MOTOR3_No018.System := W#16#0;
   MOTOR3_No018.CmdOS := W#16#0;
   MOTOR3_No018.MirrorCmdOS := W#16#0;
   MOTOR3_No018.Test := W#16#0;
   MOTOR3_No018.AlarmOS := W#16#0;
   MOTOR3_No018.StatusOS := W#16#0;
   MOTOR3_No018.SysStatusOS := W#16#0;
   MOTOR3_No018.Status1 := W#16#0;
   MOTOR3_No018.Status2 := W#16#0;
   MOTOR3_No018.Status3 := B#16#0;
   MOTOR3_No018.InputEdges := B#16#0;
   MOTOR3_No018.AutoEdges := W#16#0;
   MOTOR3_No018.DataTimeExtFault.StartTime := L#0;
   MOTOR3_No018.DataTimeExtFault.StartEdge := FALSE;
   MOTOR3_No018.DataTimeFeedback.StartTime := L#0;
   MOTOR3_No018.DataTimeFeedback.StartEdge := FALSE;
   MOTOR3_No018.DataTimeActFault.StartTime := L#0;
   MOTOR3_No018.DataTimeActFault.StartEdge := FALSE;
   MOTOR3_No018.DataTimeAutoAl.StartTime := L#0;
   MOTOR3_No018.DataTimeAutoAl.StartEdge := FALSE;
   MOTOR3_No018.DataTimeRestart.StartTime := L#0;
   MOTOR3_No018.DataTimeRestart.StartEdge := FALSE;
   MOTOR3_No018.DataTimeChgSF.StartTime := L#0;
   MOTOR3_No018.DataTimeChgSF.StartEdge := FALSE;
   MOTOR3_No018.DataTimeChgFS.StartTime := L#0;
   MOTOR3_No018.DataTimeChgFS.StartEdge := FALSE;
   MOTOR3_No018.DataTimeChgDirec.StartTime := L#0;
   MOTOR3_No018.DataTimeChgDirec.StartEdge := FALSE;
   MOTOR3_No018.PCONF.Modeswitches.M0_ConstantOut := FALSE;
   MOTOR3_No018.PCONF.Modeswitches.M1_AutoManLoc := FALSE;
   MOTOR3_No018.PCONF.Modeswitches.M2_NoActFeedFault := FALSE;
   MOTOR3_No018.PCONF.Modeswitches.M3_NoStopIfFault := FALSE;
   MOTOR3_No018.PCONF.Modeswitches.M4_RestrtAftBlack := FALSE;
   MOTOR3_No018.PCONF.Modeswitches.M5_ResetOSonly := FALSE;
   MOTOR3_No018.PCONF.Modeswitches.sw06 := FALSE;
   MOTOR3_No018.PCONF.Modeswitches.M7_ChgSFviaStop := FALSE;
   MOTOR3_No018.PCONF.Modeswitches.M8_ChgFSviaStop := FALSE;
   MOTOR3_No018.PCONF.Modeswitches.M9_StopIfAutoFail := FALSE;
   MOTOR3_No018.PCONF.Modeswitches.M10_ExtFaultNC := FALSE;
   MOTOR3_No018.PCONF.Modeswitches.sw11 := FALSE;
   MOTOR3_No018.PCONF.Modeswitches.sw12 := FALSE;
   MOTOR3_No018.PCONF.Modeswitches.sw13 := FALSE;
   MOTOR3_No018.PCONF.Modeswitches.sw14 := FALSE;
   MOTOR3_No018.PCONF.Modeswitches.sw15 := FALSE;
   MOTOR3_No018.PCONF.DlyTExtFault := T#0MS;
   MOTOR3_No018.PCONF.DlyTFeedback := T#0MS;
   MOTOR3_No018.PCONF.DlyTActFault := T#0MS;
   MOTOR3_No018.PCONF.DlyTAutoAl := T#0MS;
   MOTOR3_No018.PCONF.DlyTRestart := T#0MS;
   MOTOR3_No018.PCONF.DlyTChgSF := T#0MS;
   MOTOR3_No018.PCONF.DlyTChgFS := T#0MS;
   MOTOR3_No018.PCONF.DlyTChgDirec := T#0MS;
   MOTOR3_No019.System := W#16#0;
   MOTOR3_No019.CmdOS := W#16#0;
   MOTOR3_No019.MirrorCmdOS := W#16#0;
   MOTOR3_No019.Test := W#16#0;
   MOTOR3_No019.AlarmOS := W#16#0;
   MOTOR3_No019.StatusOS := W#16#0;
   MOTOR3_No019.SysStatusOS := W#16#0;
   MOTOR3_No019.Status1 := W#16#0;
   MOTOR3_No019.Status2 := W#16#0;
   MOTOR3_No019.Status3 := B#16#0;
   MOTOR3_No019.InputEdges := B#16#0;
   MOTOR3_No019.AutoEdges := W#16#0;
   MOTOR3_No019.DataTimeExtFault.StartTime := L#0;
   MOTOR3_No019.DataTimeExtFault.StartEdge := FALSE;
   MOTOR3_No019.DataTimeFeedback.StartTime := L#0;
   MOTOR3_No019.DataTimeFeedback.StartEdge := FALSE;
   MOTOR3_No019.DataTimeActFault.StartTime := L#0;
   MOTOR3_No019.DataTimeActFault.StartEdge := FALSE;
   MOTOR3_No019.DataTimeAutoAl.StartTime := L#0;
   MOTOR3_No019.DataTimeAutoAl.StartEdge := FALSE;
   MOTOR3_No019.DataTimeRestart.StartTime := L#0;
   MOTOR3_No019.DataTimeRestart.StartEdge := FALSE;
   MOTOR3_No019.DataTimeChgSF.StartTime := L#0;
   MOTOR3_No019.DataTimeChgSF.StartEdge := FALSE;
   MOTOR3_No019.DataTimeChgFS.StartTime := L#0;
   MOTOR3_No019.DataTimeChgFS.StartEdge := FALSE;
   MOTOR3_No019.DataTimeChgDirec.StartTime := L#0;
   MOTOR3_No019.DataTimeChgDirec.StartEdge := FALSE;
   MOTOR3_No019.PCONF.Modeswitches.M0_ConstantOut := FALSE;
   MOTOR3_No019.PCONF.Modeswitches.M1_AutoManLoc := FALSE;
   MOTOR3_No019.PCONF.Modeswitches.M2_NoActFeedFault := FALSE;
   MOTOR3_No019.PCONF.Modeswitches.M3_NoStopIfFault := FALSE;
   MOTOR3_No019.PCONF.Modeswitches.M4_RestrtAftBlack := FALSE;
   MOTOR3_No019.PCONF.Modeswitches.M5_ResetOSonly := FALSE;
   MOTOR3_No019.PCONF.Modeswitches.sw06 := FALSE;
   MOTOR3_No019.PCONF.Modeswitches.M7_ChgSFviaStop := FALSE;
   MOTOR3_No019.PCONF.Modeswitches.M8_ChgFSviaStop := FALSE;
   MOTOR3_No019.PCONF.Modeswitches.M9_StopIfAutoFail := FALSE;
   MOTOR3_No019.PCONF.Modeswitches.M10_ExtFaultNC := FALSE;
   MOTOR3_No019.PCONF.Modeswitches.sw11 := FALSE;
   MOTOR3_No019.PCONF.Modeswitches.sw12 := FALSE;
   MOTOR3_No019.PCONF.Modeswitches.sw13 := FALSE;
   MOTOR3_No019.PCONF.Modeswitches.sw14 := FALSE;
   MOTOR3_No019.PCONF.Modeswitches.sw15 := FALSE;
   MOTOR3_No019.PCONF.DlyTExtFault := T#0MS;
   MOTOR3_No019.PCONF.DlyTFeedback := T#0MS;
   MOTOR3_No019.PCONF.DlyTActFault := T#0MS;
   MOTOR3_No019.PCONF.DlyTAutoAl := T#0MS;
   MOTOR3_No019.PCONF.DlyTRestart := T#0MS;
   MOTOR3_No019.PCONF.DlyTChgSF := T#0MS;
   MOTOR3_No019.PCONF.DlyTChgFS := T#0MS;
   MOTOR3_No019.PCONF.DlyTChgDirec := T#0MS;
   MOTOR3_No020.System := W#16#0;
   MOTOR3_No020.CmdOS := W#16#0;
   MOTOR3_No020.MirrorCmdOS := W#16#0;
   MOTOR3_No020.Test := W#16#0;
   MOTOR3_No020.AlarmOS := W#16#0;
   MOTOR3_No020.StatusOS := W#16#0;
   MOTOR3_No020.SysStatusOS := W#16#0;
   MOTOR3_No020.Status1 := W#16#0;
   MOTOR3_No020.Status2 := W#16#0;
   MOTOR3_No020.Status3 := B#16#0;
   MOTOR3_No020.InputEdges := B#16#0;
   MOTOR3_No020.AutoEdges := W#16#0;
   MOTOR3_No020.DataTimeExtFault.StartTime := L#0;
   MOTOR3_No020.DataTimeExtFault.StartEdge := FALSE;
   MOTOR3_No020.DataTimeFeedback.StartTime := L#0;
   MOTOR3_No020.DataTimeFeedback.StartEdge := FALSE;
   MOTOR3_No020.DataTimeActFault.StartTime := L#0;
   MOTOR3_No020.DataTimeActFault.StartEdge := FALSE;
   MOTOR3_No020.DataTimeAutoAl.StartTime := L#0;
   MOTOR3_No020.DataTimeAutoAl.StartEdge := FALSE;
   MOTOR3_No020.DataTimeRestart.StartTime := L#0;
   MOTOR3_No020.DataTimeRestart.StartEdge := FALSE;
   MOTOR3_No020.DataTimeChgSF.StartTime := L#0;
   MOTOR3_No020.DataTimeChgSF.StartEdge := FALSE;
   MOTOR3_No020.DataTimeChgFS.StartTime := L#0;
   MOTOR3_No020.DataTimeChgFS.StartEdge := FALSE;
   MOTOR3_No020.DataTimeChgDirec.StartTime := L#0;
   MOTOR3_No020.DataTimeChgDirec.StartEdge := FALSE;
   MOTOR3_No020.PCONF.Modeswitches.M0_ConstantOut := FALSE;
   MOTOR3_No020.PCONF.Modeswitches.M1_AutoManLoc := FALSE;
   MOTOR3_No020.PCONF.Modeswitches.M2_NoActFeedFault := FALSE;
   MOTOR3_No020.PCONF.Modeswitches.M3_NoStopIfFault := FALSE;
   MOTOR3_No020.PCONF.Modeswitches.M4_RestrtAftBlack := FALSE;
   MOTOR3_No020.PCONF.Modeswitches.M5_ResetOSonly := FALSE;
   MOTOR3_No020.PCONF.Modeswitches.sw06 := FALSE;
   MOTOR3_No020.PCONF.Modeswitches.M7_ChgSFviaStop := FALSE;
   MOTOR3_No020.PCONF.Modeswitches.M8_ChgFSviaStop := FALSE;
   MOTOR3_No020.PCONF.Modeswitches.M9_StopIfAutoFail := FALSE;
   MOTOR3_No020.PCONF.Modeswitches.M10_ExtFaultNC := FALSE;
   MOTOR3_No020.PCONF.Modeswitches.sw11 := FALSE;
   MOTOR3_No020.PCONF.Modeswitches.sw12 := FALSE;
   MOTOR3_No020.PCONF.Modeswitches.sw13 := FALSE;
   MOTOR3_No020.PCONF.Modeswitches.sw14 := FALSE;
   MOTOR3_No020.PCONF.Modeswitches.sw15 := FALSE;
   MOTOR3_No020.PCONF.DlyTExtFault := T#0MS;
   MOTOR3_No020.PCONF.DlyTFeedback := T#0MS;
   MOTOR3_No020.PCONF.DlyTActFault := T#0MS;
   MOTOR3_No020.PCONF.DlyTAutoAl := T#0MS;
   MOTOR3_No020.PCONF.DlyTRestart := T#0MS;
   MOTOR3_No020.PCONF.DlyTChgSF := T#0MS;
   MOTOR3_No020.PCONF.DlyTChgFS := T#0MS;
   MOTOR3_No020.PCONF.DlyTChgDirec := T#0MS;
   MOTOR3_No021.System := W#16#0;
   MOTOR3_No021.CmdOS := W#16#0;
   MOTOR3_No021.MirrorCmdOS := W#16#0;
   MOTOR3_No021.Test := W#16#0;
   MOTOR3_No021.AlarmOS := W#16#0;
   MOTOR3_No021.StatusOS := W#16#0;
   MOTOR3_No021.SysStatusOS := W#16#0;
   MOTOR3_No021.Status1 := W#16#0;
   MOTOR3_No021.Status2 := W#16#0;
   MOTOR3_No021.Status3 := B#16#0;
   MOTOR3_No021.InputEdges := B#16#0;
   MOTOR3_No021.AutoEdges := W#16#0;
   MOTOR3_No021.DataTimeExtFault.StartTime := L#0;
   MOTOR3_No021.DataTimeExtFault.StartEdge := FALSE;
   MOTOR3_No021.DataTimeFeedback.StartTime := L#0;
   MOTOR3_No021.DataTimeFeedback.StartEdge := FALSE;
   MOTOR3_No021.DataTimeActFault.StartTime := L#0;
   MOTOR3_No021.DataTimeActFault.StartEdge := FALSE;
   MOTOR3_No021.DataTimeAutoAl.StartTime := L#0;
   MOTOR3_No021.DataTimeAutoAl.StartEdge := FALSE;
   MOTOR3_No021.DataTimeRestart.StartTime := L#0;
   MOTOR3_No021.DataTimeRestart.StartEdge := FALSE;
   MOTOR3_No021.DataTimeChgSF.StartTime := L#0;
   MOTOR3_No021.DataTimeChgSF.StartEdge := FALSE;
   MOTOR3_No021.DataTimeChgFS.StartTime := L#0;
   MOTOR3_No021.DataTimeChgFS.StartEdge := FALSE;
   MOTOR3_No021.DataTimeChgDirec.StartTime := L#0;
   MOTOR3_No021.DataTimeChgDirec.StartEdge := FALSE;
   MOTOR3_No021.PCONF.Modeswitches.M0_ConstantOut := FALSE;
   MOTOR3_No021.PCONF.Modeswitches.M1_AutoManLoc := FALSE;
   MOTOR3_No021.PCONF.Modeswitches.M2_NoActFeedFault := FALSE;
   MOTOR3_No021.PCONF.Modeswitches.M3_NoStopIfFault := FALSE;
   MOTOR3_No021.PCONF.Modeswitches.M4_RestrtAftBlack := FALSE;
   MOTOR3_No021.PCONF.Modeswitches.M5_ResetOSonly := FALSE;
   MOTOR3_No021.PCONF.Modeswitches.sw06 := FALSE;
   MOTOR3_No021.PCONF.Modeswitches.M7_ChgSFviaStop := FALSE;
   MOTOR3_No021.PCONF.Modeswitches.M8_ChgFSviaStop := FALSE;
   MOTOR3_No021.PCONF.Modeswitches.M9_StopIfAutoFail := FALSE;
   MOTOR3_No021.PCONF.Modeswitches.M10_ExtFaultNC := FALSE;
   MOTOR3_No021.PCONF.Modeswitches.sw11 := FALSE;
   MOTOR3_No021.PCONF.Modeswitches.sw12 := FALSE;
   MOTOR3_No021.PCONF.Modeswitches.sw13 := FALSE;
   MOTOR3_No021.PCONF.Modeswitches.sw14 := FALSE;
   MOTOR3_No021.PCONF.Modeswitches.sw15 := FALSE;
   MOTOR3_No021.PCONF.DlyTExtFault := T#0MS;
   MOTOR3_No021.PCONF.DlyTFeedback := T#0MS;
   MOTOR3_No021.PCONF.DlyTActFault := T#0MS;
   MOTOR3_No021.PCONF.DlyTAutoAl := T#0MS;
   MOTOR3_No021.PCONF.DlyTRestart := T#0MS;
   MOTOR3_No021.PCONF.DlyTChgSF := T#0MS;
   MOTOR3_No021.PCONF.DlyTChgFS := T#0MS;
   MOTOR3_No021.PCONF.DlyTChgDirec := T#0MS;
   MOTOR3_No022.System := W#16#0;
   MOTOR3_No022.CmdOS := W#16#0;
   MOTOR3_No022.MirrorCmdOS := W#16#0;
   MOTOR3_No022.Test := W#16#0;
   MOTOR3_No022.AlarmOS := W#16#0;
   MOTOR3_No022.StatusOS := W#16#0;
   MOTOR3_No022.SysStatusOS := W#16#0;
   MOTOR3_No022.Status1 := W#16#0;
   MOTOR3_No022.Status2 := W#16#0;
   MOTOR3_No022.Status3 := B#16#0;
   MOTOR3_No022.InputEdges := B#16#0;
   MOTOR3_No022.AutoEdges := W#16#0;
   MOTOR3_No022.DataTimeExtFault.StartTime := L#0;
   MOTOR3_No022.DataTimeExtFault.StartEdge := FALSE;
   MOTOR3_No022.DataTimeFeedback.StartTime := L#0;
   MOTOR3_No022.DataTimeFeedback.StartEdge := FALSE;
   MOTOR3_No022.DataTimeActFault.StartTime := L#0;
   MOTOR3_No022.DataTimeActFault.StartEdge := FALSE;
   MOTOR3_No022.DataTimeAutoAl.StartTime := L#0;
   MOTOR3_No022.DataTimeAutoAl.StartEdge := FALSE;
   MOTOR3_No022.DataTimeRestart.StartTime := L#0;
   MOTOR3_No022.DataTimeRestart.StartEdge := FALSE;
   MOTOR3_No022.DataTimeChgSF.StartTime := L#0;
   MOTOR3_No022.DataTimeChgSF.StartEdge := FALSE;
   MOTOR3_No022.DataTimeChgFS.StartTime := L#0;
   MOTOR3_No022.DataTimeChgFS.StartEdge := FALSE;
   MOTOR3_No022.DataTimeChgDirec.StartTime := L#0;
   MOTOR3_No022.DataTimeChgDirec.StartEdge := FALSE;
   MOTOR3_No022.PCONF.Modeswitches.M0_ConstantOut := FALSE;
   MOTOR3_No022.PCONF.Modeswitches.M1_AutoManLoc := FALSE;
   MOTOR3_No022.PCONF.Modeswitches.M2_NoActFeedFault := FALSE;
   MOTOR3_No022.PCONF.Modeswitches.M3_NoStopIfFault := FALSE;
   MOTOR3_No022.PCONF.Modeswitches.M4_RestrtAftBlack := FALSE;
   MOTOR3_No022.PCONF.Modeswitches.M5_ResetOSonly := FALSE;
   MOTOR3_No022.PCONF.Modeswitches.sw06 := FALSE;
   MOTOR3_No022.PCONF.Modeswitches.M7_ChgSFviaStop := FALSE;
   MOTOR3_No022.PCONF.Modeswitches.M8_ChgFSviaStop := FALSE;
   MOTOR3_No022.PCONF.Modeswitches.M9_StopIfAutoFail := FALSE;
   MOTOR3_No022.PCONF.Modeswitches.M10_ExtFaultNC := FALSE;
   MOTOR3_No022.PCONF.Modeswitches.sw11 := FALSE;
   MOTOR3_No022.PCONF.Modeswitches.sw12 := FALSE;
   MOTOR3_No022.PCONF.Modeswitches.sw13 := FALSE;
   MOTOR3_No022.PCONF.Modeswitches.sw14 := FALSE;
   MOTOR3_No022.PCONF.Modeswitches.sw15 := FALSE;
   MOTOR3_No022.PCONF.DlyTExtFault := T#0MS;
   MOTOR3_No022.PCONF.DlyTFeedback := T#0MS;
   MOTOR3_No022.PCONF.DlyTActFault := T#0MS;
   MOTOR3_No022.PCONF.DlyTAutoAl := T#0MS;
   MOTOR3_No022.PCONF.DlyTRestart := T#0MS;
   MOTOR3_No022.PCONF.DlyTChgSF := T#0MS;
   MOTOR3_No022.PCONF.DlyTChgFS := T#0MS;
   MOTOR3_No022.PCONF.DlyTChgDirec := T#0MS;
   MOTOR3_No023.System := W#16#0;
   MOTOR3_No023.CmdOS := W#16#0;
   MOTOR3_No023.MirrorCmdOS := W#16#0;
   MOTOR3_No023.Test := W#16#0;
   MOTOR3_No023.AlarmOS := W#16#0;
   MOTOR3_No023.StatusOS := W#16#0;
   MOTOR3_No023.SysStatusOS := W#16#0;
   MOTOR3_No023.Status1 := W#16#0;
   MOTOR3_No023.Status2 := W#16#0;
   MOTOR3_No023.Status3 := B#16#0;
   MOTOR3_No023.InputEdges := B#16#0;
   MOTOR3_No023.AutoEdges := W#16#0;
   MOTOR3_No023.DataTimeExtFault.StartTime := L#0;
   MOTOR3_No023.DataTimeExtFault.StartEdge := FALSE;
   MOTOR3_No023.DataTimeFeedback.StartTime := L#0;
   MOTOR3_No023.DataTimeFeedback.StartEdge := FALSE;
   MOTOR3_No023.DataTimeActFault.StartTime := L#0;
   MOTOR3_No023.DataTimeActFault.StartEdge := FALSE;
   MOTOR3_No023.DataTimeAutoAl.StartTime := L#0;
   MOTOR3_No023.DataTimeAutoAl.StartEdge := FALSE;
   MOTOR3_No023.DataTimeRestart.StartTime := L#0;
   MOTOR3_No023.DataTimeRestart.StartEdge := FALSE;
   MOTOR3_No023.DataTimeChgSF.StartTime := L#0;
   MOTOR3_No023.DataTimeChgSF.StartEdge := FALSE;
   MOTOR3_No023.DataTimeChgFS.StartTime := L#0;
   MOTOR3_No023.DataTimeChgFS.StartEdge := FALSE;
   MOTOR3_No023.DataTimeChgDirec.StartTime := L#0;
   MOTOR3_No023.DataTimeChgDirec.StartEdge := FALSE;
   MOTOR3_No023.PCONF.Modeswitches.M0_ConstantOut := FALSE;
   MOTOR3_No023.PCONF.Modeswitches.M1_AutoManLoc := FALSE;
   MOTOR3_No023.PCONF.Modeswitches.M2_NoActFeedFault := FALSE;
   MOTOR3_No023.PCONF.Modeswitches.M3_NoStopIfFault := FALSE;
   MOTOR3_No023.PCONF.Modeswitches.M4_RestrtAftBlack := FALSE;
   MOTOR3_No023.PCONF.Modeswitches.M5_ResetOSonly := FALSE;
   MOTOR3_No023.PCONF.Modeswitches.sw06 := FALSE;
   MOTOR3_No023.PCONF.Modeswitches.M7_ChgSFviaStop := FALSE;
   MOTOR3_No023.PCONF.Modeswitches.M8_ChgFSviaStop := FALSE;
   MOTOR3_No023.PCONF.Modeswitches.M9_StopIfAutoFail := FALSE;
   MOTOR3_No023.PCONF.Modeswitches.M10_ExtFaultNC := FALSE;
   MOTOR3_No023.PCONF.Modeswitches.sw11 := FALSE;
   MOTOR3_No023.PCONF.Modeswitches.sw12 := FALSE;
   MOTOR3_No023.PCONF.Modeswitches.sw13 := FALSE;
   MOTOR3_No023.PCONF.Modeswitches.sw14 := FALSE;
   MOTOR3_No023.PCONF.Modeswitches.sw15 := FALSE;
   MOTOR3_No023.PCONF.DlyTExtFault := T#0MS;
   MOTOR3_No023.PCONF.DlyTFeedback := T#0MS;
   MOTOR3_No023.PCONF.DlyTActFault := T#0MS;
   MOTOR3_No023.PCONF.DlyTAutoAl := T#0MS;
   MOTOR3_No023.PCONF.DlyTRestart := T#0MS;
   MOTOR3_No023.PCONF.DlyTChgSF := T#0MS;
   MOTOR3_No023.PCONF.DlyTChgFS := T#0MS;
   MOTOR3_No023.PCONF.DlyTChgDirec := T#0MS;
   MOTOR3_No024.System := W#16#0;
   MOTOR3_No024.CmdOS := W#16#0;
   MOTOR3_No024.MirrorCmdOS := W#16#0;
   MOTOR3_No024.Test := W#16#0;
   MOTOR3_No024.AlarmOS := W#16#0;
   MOTOR3_No024.StatusOS := W#16#0;
   MOTOR3_No024.SysStatusOS := W#16#0;
   MOTOR3_No024.Status1 := W#16#0;
   MOTOR3_No024.Status2 := W#16#0;
   MOTOR3_No024.Status3 := B#16#0;
   MOTOR3_No024.InputEdges := B#16#0;
   MOTOR3_No024.AutoEdges := W#16#0;
   MOTOR3_No024.DataTimeExtFault.StartTime := L#0;
   MOTOR3_No024.DataTimeExtFault.StartEdge := FALSE;
   MOTOR3_No024.DataTimeFeedback.StartTime := L#0;
   MOTOR3_No024.DataTimeFeedback.StartEdge := FALSE;
   MOTOR3_No024.DataTimeActFault.StartTime := L#0;
   MOTOR3_No024.DataTimeActFault.StartEdge := FALSE;
   MOTOR3_No024.DataTimeAutoAl.StartTime := L#0;
   MOTOR3_No024.DataTimeAutoAl.StartEdge := FALSE;
   MOTOR3_No024.DataTimeRestart.StartTime := L#0;
   MOTOR3_No024.DataTimeRestart.StartEdge := FALSE;
   MOTOR3_No024.DataTimeChgSF.StartTime := L#0;
   MOTOR3_No024.DataTimeChgSF.StartEdge := FALSE;
   MOTOR3_No024.DataTimeChgFS.StartTime := L#0;
   MOTOR3_No024.DataTimeChgFS.StartEdge := FALSE;
   MOTOR3_No024.DataTimeChgDirec.StartTime := L#0;
   MOTOR3_No024.DataTimeChgDirec.StartEdge := FALSE;
   MOTOR3_No024.PCONF.Modeswitches.M0_ConstantOut := FALSE;
   MOTOR3_No024.PCONF.Modeswitches.M1_AutoManLoc := FALSE;
   MOTOR3_No024.PCONF.Modeswitches.M2_NoActFeedFault := FALSE;
   MOTOR3_No024.PCONF.Modeswitches.M3_NoStopIfFault := FALSE;
   MOTOR3_No024.PCONF.Modeswitches.M4_RestrtAftBlack := FALSE;
   MOTOR3_No024.PCONF.Modeswitches.M5_ResetOSonly := FALSE;
   MOTOR3_No024.PCONF.Modeswitches.sw06 := FALSE;
   MOTOR3_No024.PCONF.Modeswitches.M7_ChgSFviaStop := FALSE;
   MOTOR3_No024.PCONF.Modeswitches.M8_ChgFSviaStop := FALSE;
   MOTOR3_No024.PCONF.Modeswitches.M9_StopIfAutoFail := FALSE;
   MOTOR3_No024.PCONF.Modeswitches.M10_ExtFaultNC := FALSE;
   MOTOR3_No024.PCONF.Modeswitches.sw11 := FALSE;
   MOTOR3_No024.PCONF.Modeswitches.sw12 := FALSE;
   MOTOR3_No024.PCONF.Modeswitches.sw13 := FALSE;
   MOTOR3_No024.PCONF.Modeswitches.sw14 := FALSE;
   MOTOR3_No024.PCONF.Modeswitches.sw15 := FALSE;
   MOTOR3_No024.PCONF.DlyTExtFault := T#0MS;
   MOTOR3_No024.PCONF.DlyTFeedback := T#0MS;
   MOTOR3_No024.PCONF.DlyTActFault := T#0MS;
   MOTOR3_No024.PCONF.DlyTAutoAl := T#0MS;
   MOTOR3_No024.PCONF.DlyTRestart := T#0MS;
   MOTOR3_No024.PCONF.DlyTChgSF := T#0MS;
   MOTOR3_No024.PCONF.DlyTChgFS := T#0MS;
   MOTOR3_No024.PCONF.DlyTChgDirec := T#0MS;
   MOTOR3_No025.System := W#16#0;
   MOTOR3_No025.CmdOS := W#16#0;
   MOTOR3_No025.MirrorCmdOS := W#16#0;
   MOTOR3_No025.Test := W#16#0;
   MOTOR3_No025.AlarmOS := W#16#0;
   MOTOR3_No025.StatusOS := W#16#0;
   MOTOR3_No025.SysStatusOS := W#16#0;
   MOTOR3_No025.Status1 := W#16#0;
   MOTOR3_No025.Status2 := W#16#0;
   MOTOR3_No025.Status3 := B#16#0;
   MOTOR3_No025.InputEdges := B#16#0;
   MOTOR3_No025.AutoEdges := W#16#0;
   MOTOR3_No025.DataTimeExtFault.StartTime := L#0;
   MOTOR3_No025.DataTimeExtFault.StartEdge := FALSE;
   MOTOR3_No025.DataTimeFeedback.StartTime := L#0;
   MOTOR3_No025.DataTimeFeedback.StartEdge := FALSE;
   MOTOR3_No025.DataTimeActFault.StartTime := L#0;
   MOTOR3_No025.DataTimeActFault.StartEdge := FALSE;
   MOTOR3_No025.DataTimeAutoAl.StartTime := L#0;
   MOTOR3_No025.DataTimeAutoAl.StartEdge := FALSE;
   MOTOR3_No025.DataTimeRestart.StartTime := L#0;
   MOTOR3_No025.DataTimeRestart.StartEdge := FALSE;
   MOTOR3_No025.DataTimeChgSF.StartTime := L#0;
   MOTOR3_No025.DataTimeChgSF.StartEdge := FALSE;
   MOTOR3_No025.DataTimeChgFS.StartTime := L#0;
   MOTOR3_No025.DataTimeChgFS.StartEdge := FALSE;
   MOTOR3_No025.DataTimeChgDirec.StartTime := L#0;
   MOTOR3_No025.DataTimeChgDirec.StartEdge := FALSE;
   MOTOR3_No025.PCONF.Modeswitches.M0_ConstantOut := FALSE;
   MOTOR3_No025.PCONF.Modeswitches.M1_AutoManLoc := FALSE;
   MOTOR3_No025.PCONF.Modeswitches.M2_NoActFeedFault := FALSE;
   MOTOR3_No025.PCONF.Modeswitches.M3_NoStopIfFault := FALSE;
   MOTOR3_No025.PCONF.Modeswitches.M4_RestrtAftBlack := FALSE;
   MOTOR3_No025.PCONF.Modeswitches.M5_ResetOSonly := FALSE;
   MOTOR3_No025.PCONF.Modeswitches.sw06 := FALSE;
   MOTOR3_No025.PCONF.Modeswitches.M7_ChgSFviaStop := FALSE;
   MOTOR3_No025.PCONF.Modeswitches.M8_ChgFSviaStop := FALSE;
   MOTOR3_No025.PCONF.Modeswitches.M9_StopIfAutoFail := FALSE;
   MOTOR3_No025.PCONF.Modeswitches.M10_ExtFaultNC := FALSE;
   MOTOR3_No025.PCONF.Modeswitches.sw11 := FALSE;
   MOTOR3_No025.PCONF.Modeswitches.sw12 := FALSE;
   MOTOR3_No025.PCONF.Modeswitches.sw13 := FALSE;
   MOTOR3_No025.PCONF.Modeswitches.sw14 := FALSE;
   MOTOR3_No025.PCONF.Modeswitches.sw15 := FALSE;
   MOTOR3_No025.PCONF.DlyTExtFault := T#0MS;
   MOTOR3_No025.PCONF.DlyTFeedback := T#0MS;
   MOTOR3_No025.PCONF.DlyTActFault := T#0MS;
   MOTOR3_No025.PCONF.DlyTAutoAl := T#0MS;
   MOTOR3_No025.PCONF.DlyTRestart := T#0MS;
   MOTOR3_No025.PCONF.DlyTChgSF := T#0MS;
   MOTOR3_No025.PCONF.DlyTChgFS := T#0MS;
   MOTOR3_No025.PCONF.DlyTChgDirec := T#0MS;
END_DATA_BLOCK

